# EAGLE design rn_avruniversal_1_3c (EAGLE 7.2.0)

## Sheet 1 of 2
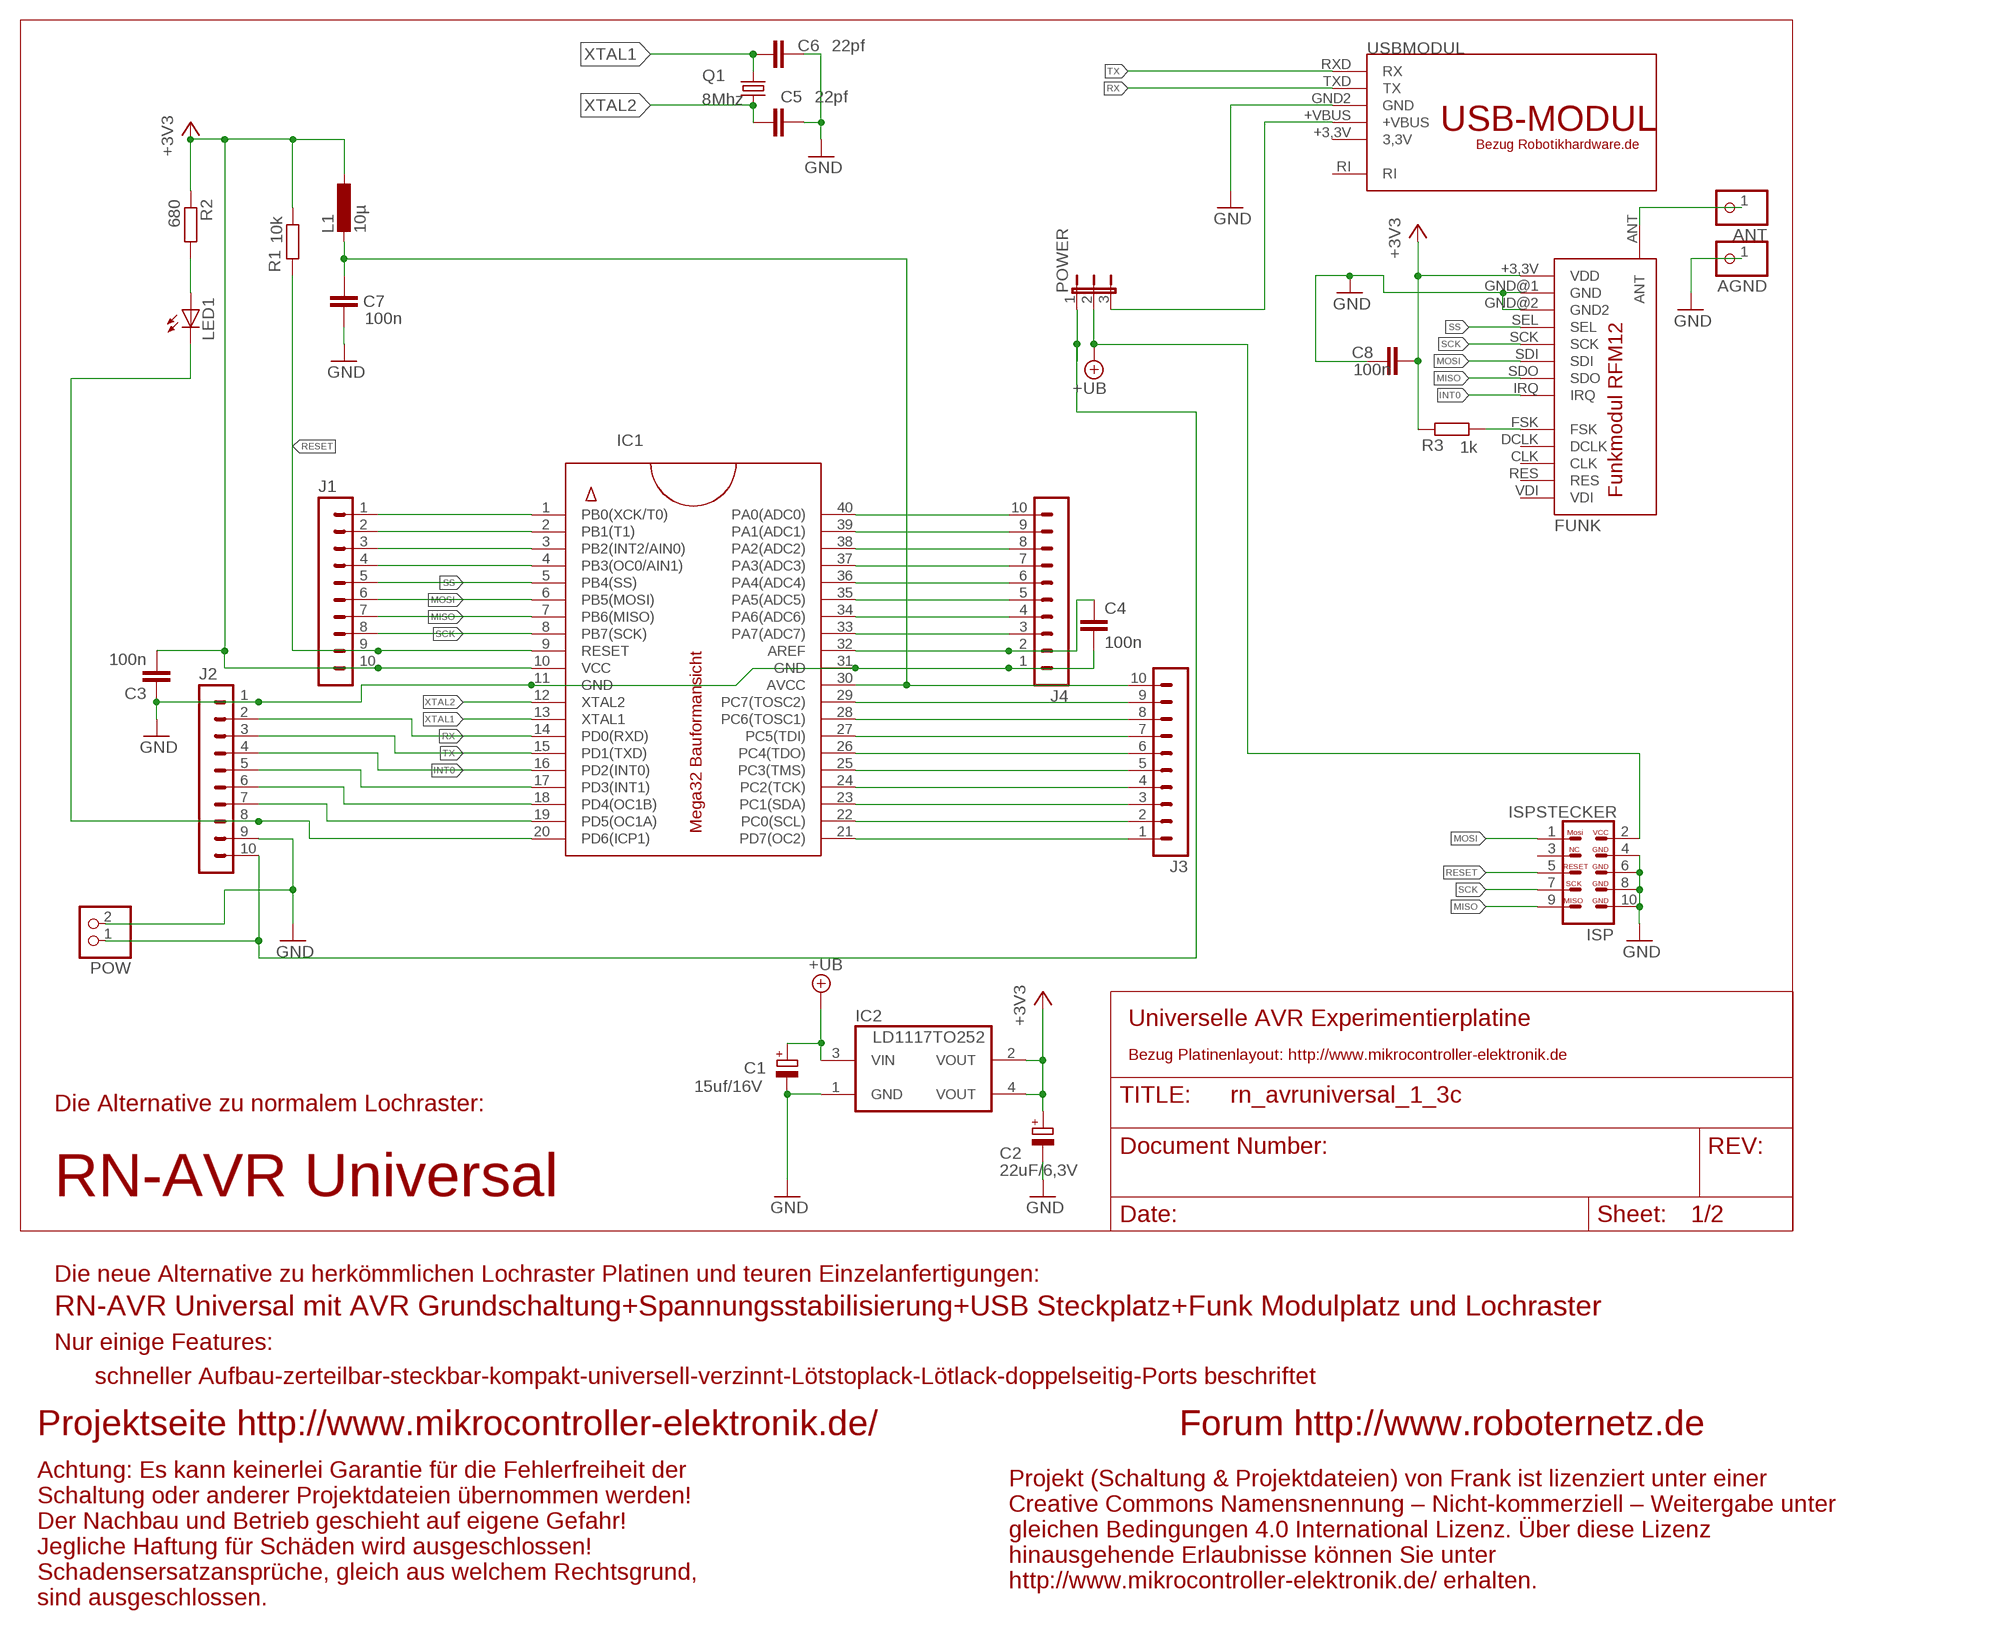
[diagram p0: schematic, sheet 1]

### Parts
AGND  PINHD-1X1  [1X01]
ANT  PINHD-1X1  [1X01]
C1  15uf/16V  CPOL-EUSMCC  [SMC_C]
C2  22uF/6,3V  CPOL-EUSMCC  [SMC_C]
C3  100n  C-EU050-024X044  [C050-024X044]
C4  100n  C-EU050-024X044  [C050-024X044]
C5  22pf  C-EU050-024X044  [C050-024X044]
C6  22pf  C-EU050-024X044  [C050-024X044]
C7  100n  C-EU050-024X044  [C050-024X044]
C8  100n  C-EU050-024X044  [C050-024X044]
FUNK  RFM12  [RFM12_SMD]
IC1  MEGA32BAUFORM  [DIL40]
IC2  LD1117TO252  [TO252]
ISP  ISPSTECKER  [ML10]
J1  AST021-10AST021-10PIN  [AST021-10PIN]
J2  AST021-10AST021-10PIN  [AST021-10PIN]
J3  AST021-10AST021-10PIN  [AST021-10PIN]
J4  AST021-10AST021-10PIN  [AST021-10PIN]
L1  10µ  L-EU0207/12  [0207/12]
LED1  LED3MM  [LED3MM]
POW  PINHD-1X2  [1X02]
POWER  JP2E  [JP2]
Q1  8Mhz  CRYTALHC49S  [HC49/S]
R1  10k  R-EU_0207/10  [0207/10]
R2  680  R-EU_0207/10  [0207/10]
R3  1k  R-EU_0207/10  [0207/10]
USBMODUL  USBMODUL_RN_BUCHSE  [USBMODUL_RN_STECKER]

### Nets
+3V3 [Power]: C2.+ C3.2 C8.2 FUNK.+3,3V(VDD) IC1.10(VCC) IC2.2(VOUT) IC2.4(VOUT) J1.10 L1.1 R1.1 R2.1 R3.2
+UB [Power]: C1.+ IC2.3(VIN) ISP.2 POWER.2
AREF: C4.1 IC1.32(AREF) J4.2
AVCC: C7.2 IC1.30(AVCC) J3.10 L1.2
GND [Power]: AGND.1 C1.- C2.- C3.1 C4.2 C5.1 C6.1 C7.1 C8.1 FUNK.GND@1(GND) FUNK.GND@2(GND2) IC1.11(GND) IC1.31(GND) IC2.1(GND) ISP.4 ISP.6 ISP.8 ISP.10 J2.1 J2.9 J4.1 POW.2 USBMODUL.GND2(GND)
INT0: FUNK.IRQ IC1.16(PD2(INT0)) J2.4
INT1: IC1.17(PD3(INT1)) J2.5
MISO: FUNK.SDO IC1.7(PB6(MISO)) ISP.9 J1.7
MOSI: FUNK.SDI IC1.6(PB5(MOSI)) ISP.1 J1.6
N$1: ANT.1 FUNK.ANT
N$2: FUNK.FSK R3.1
N$4 [Power]: POWER.3 USBMODUL.+VBUS
N$6: LED1.A R2.2
PA0: IC1.40(PA0(ADC0)) J4.10
PA1: IC1.39(PA1(ADC1)) J4.9
PA2: IC1.38(PA2(ADC2)) J4.8
PA3: IC1.37(PA3(ADC3)) J4.7
PA4: IC1.36(PA4(ADC4)) J4.6
PA5: IC1.35(PA5(ADC5)) J4.5
PA6: IC1.34(PA6(ADC6)) J4.4
PA7: IC1.33(PA7(ADC7)) J4.3
PB0: IC1.1(PB0(XCK/T0)) J1.1
PB1: IC1.2(PB1(T1)) J1.2
PB2: IC1.3(PB2(INT2/AIN0)) J1.3
PB3: IC1.4(PB3(OC0/AIN1)) J1.4
PC2: IC1.24(PC2(TCK)) J3.4
PC3: IC1.25(PC3(TMS)) J3.5
PC4: IC1.26(PC4(TDO)) J3.6
PC5: IC1.27(PC5(TDI)) J3.7
PC6: IC1.28(PC6(TOSC1)) J3.8
PC7: IC1.29(PC7(TOSC2)) J3.9
PD4: IC1.18(PD4(OC1B)) J2.6
PD5: IC1.19(PD5(OC1A)) J2.7
PD6: IC1.20(PD6(ICP1)) J2.8 LED1.K(C)
PD7: IC1.21(PD7(OC2)) J3.1
RESET: IC1.9(RESET) ISP.5 J1.9 R1.2
RX: IC1.14(PD0(RXD)) J2.2 USBMODUL.TXD(TX)
SCK: FUNK.SCK IC1.8(PB7(SCK)) ISP.7 J1.8
SCL: IC1.22(PC0(SCL)) J3.2
SDA: IC1.23(PC1(SDA)) J3.3
SS: FUNK.SEL IC1.5(PB4(SS)) J1.5
TX: IC1.15(PD1(TXD)) J2.3 USBMODUL.RXD(RX)
UEINGANG [Power]: J2.10 POW.1 POWER.1
XTAL1: C6.2 IC1.13(XTAL1) Q1.1
XTAL2: C5.2 IC1.12(XTAL2) Q1.2
Unconnected: FUNK.CLK FUNK.DCLK FUNK.RES FUNK.VDI ISP.3 USBMODUL.RI

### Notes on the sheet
- Universelle AVR Experimentierplatine
- Bezug Platinenlayout: http://www.mikrocontroller-elektronik.de
- Die Alternative zu normalem Lochraster:
- RN-AVR Universal
- Die neue Alternative zu herkömmlichen Lochraster Platinen und teuren Einzelanfertigungen:
- RN-AVR Universal mit AVR Grundschaltung+Spannungsstabilisierung+USB Steckplatz+Funk Modulplatz und Lochraster
- Nur einige Features:
- schneller Aufbau-zerteilbar-steckbar-kompakt-universell-verzinnt-Lötstoplack-Lötlack-doppelseitig-Ports beschriftet
- Projektseite http://www.mikrocontroller-elektronik.de/ | Forum http://www.roboternetz.de
- Projekt (Schaltung & Projektdateien) von Frank ist lizenziert unter einer
  Creative Commons Namensnennung – Nicht-kommerziell – Weitergabe unter
  gleichen Bedingungen 4.0 International Lizenz. Über diese Lizenz
  hinausgehende Erlaubnisse können Sie unter
  http://www.mikrocontroller-elektronik.de/ erhalten.
- Achtung: Es kann keinerlei Garantie für die Fehlerfreiheit der
  Schaltung oder anderer Projektdateien übernommen werden!
  Der Nachbau und Betrieb geschieht auf eigene Gefahr! 
  Jegliche Haftung für Schäden wird ausgeschlossen!
  Schadensersatzansprüche, gleich aus welchem Rechtsgrund,
  sind ausgeschlossen.

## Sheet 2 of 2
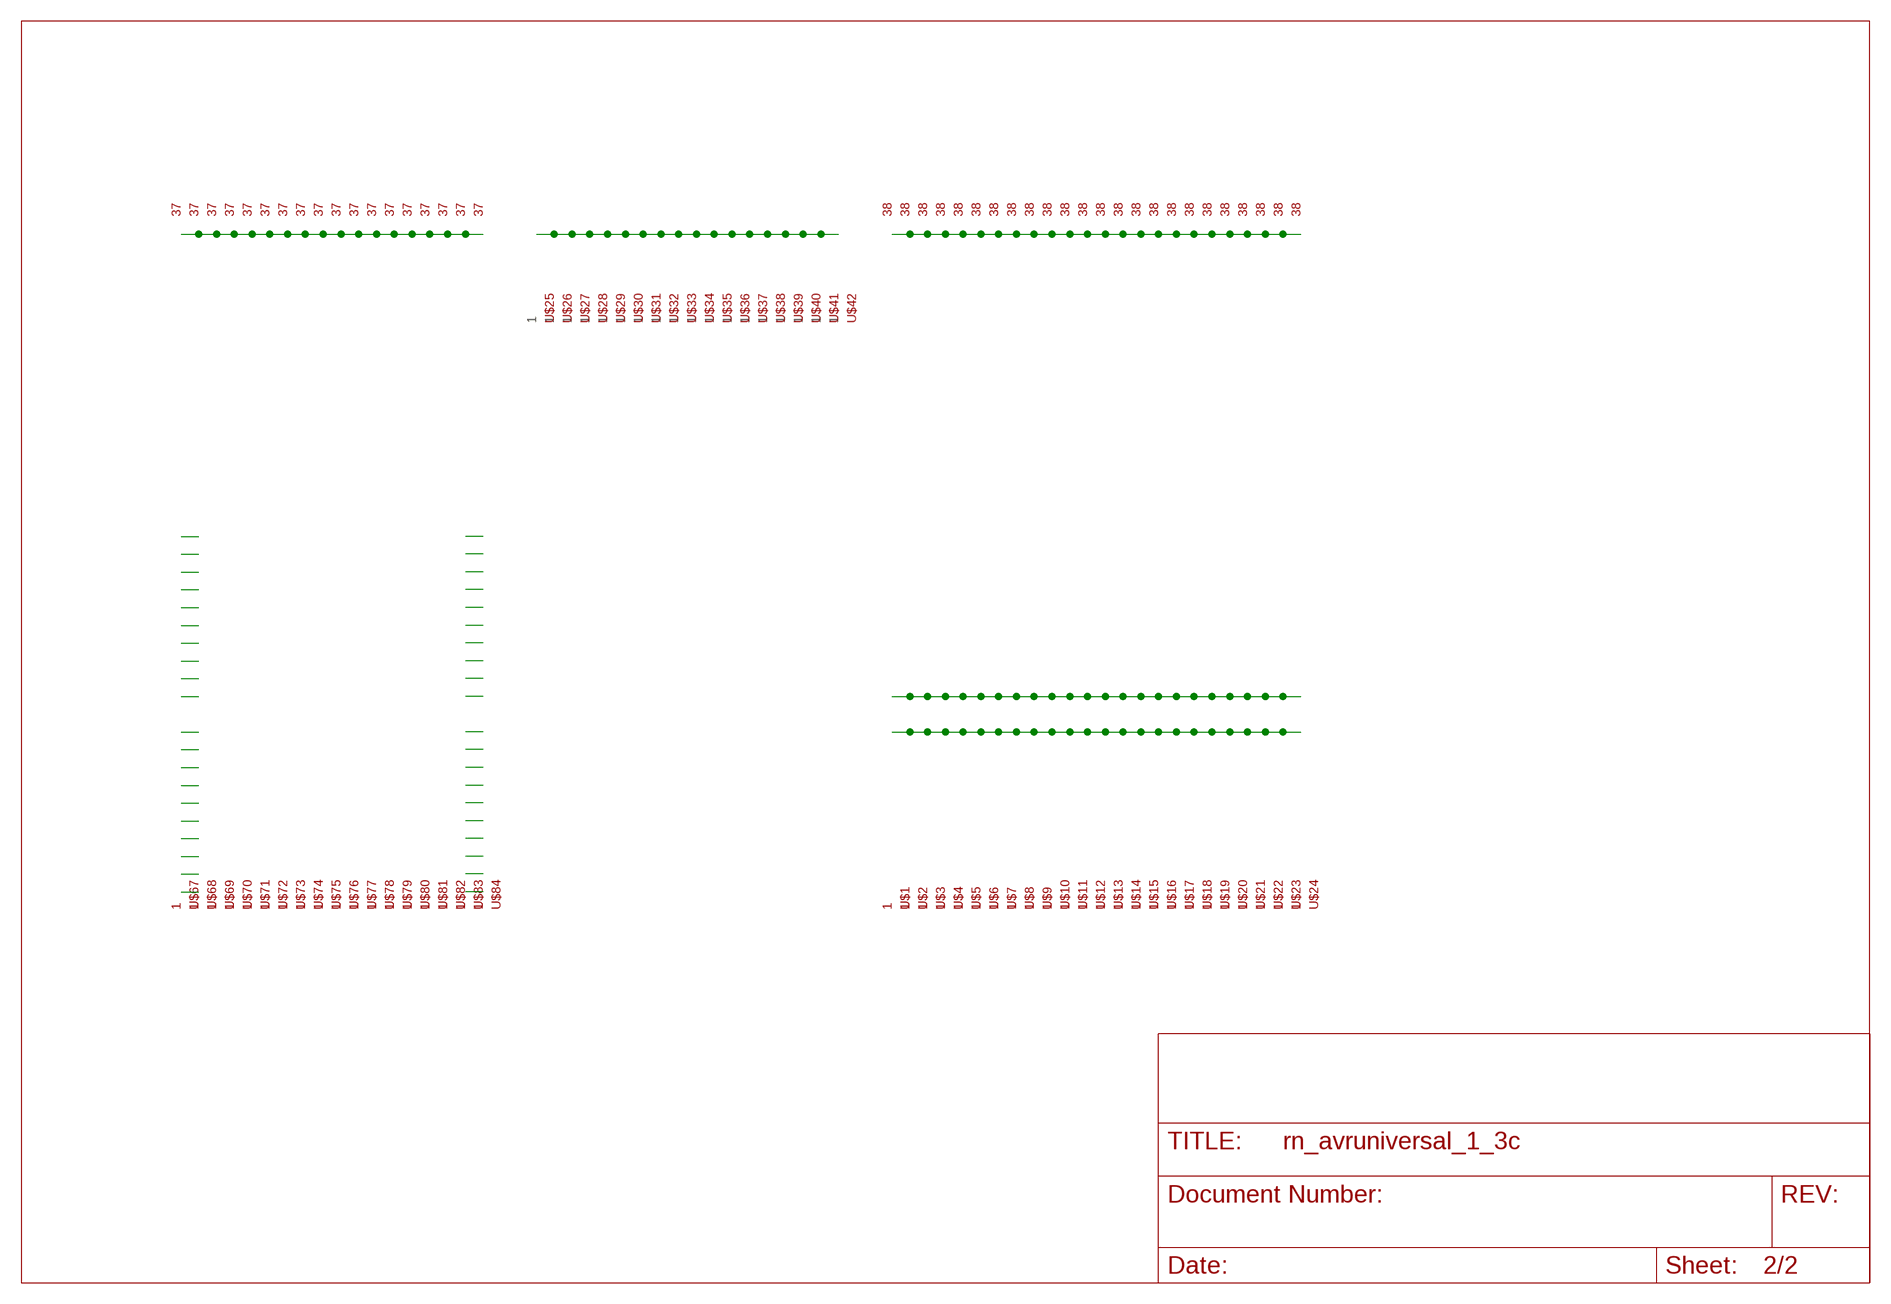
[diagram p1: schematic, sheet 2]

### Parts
U$1  LOCHRASTER38PIN  [LOCHRASTER38PIN]
U$2  LOCHRASTER38PIN  [LOCHRASTER38PIN]
U$3  LOCHRASTER38PIN  [LOCHRASTER38PIN]
U$4  LOCHRASTER38PIN  [LOCHRASTER38PIN]
U$5  LOCHRASTER38PIN  [LOCHRASTER38PIN]
U$6  LOCHRASTER38PIN  [LOCHRASTER38PIN]
U$7  LOCHRASTER38PIN  [LOCHRASTER38PIN]
U$8  LOCHRASTER38PIN  [LOCHRASTER38PIN]
U$9  LOCHRASTER38PIN  [LOCHRASTER38PIN]
U$10  LOCHRASTER38PIN  [LOCHRASTER38PIN]
U$11  LOCHRASTER38PIN  [LOCHRASTER38PIN]
U$12  LOCHRASTER38PIN  [LOCHRASTER38PIN]
U$13  LOCHRASTER38PIN  [LOCHRASTER38PIN]
U$14  LOCHRASTER38PIN  [LOCHRASTER38PIN]
U$15  LOCHRASTER38PIN  [LOCHRASTER38PIN]
U$16  LOCHRASTER38PIN  [LOCHRASTER38PIN]
U$17  LOCHRASTER38PIN  [LOCHRASTER38PIN]
U$18  LOCHRASTER38PIN  [LOCHRASTER38PIN]
U$19  LOCHRASTER38PIN  [LOCHRASTER38PIN]
U$20  LOCHRASTER38PIN  [LOCHRASTER38PIN]
U$21  LOCHRASTER38PIN  [LOCHRASTER38PIN]
U$22  LOCHRASTER38PIN  [LOCHRASTER38PIN]
U$23  LOCHRASTER38PIN  [LOCHRASTER38PIN]
U$24  LOCHRASTER38PIN  [LOCHRASTER38PIN]
U$25  LOCHRASTER5PIN  [LOACHRASTER5PIN]
U$26  LOCHRASTER5PIN  [LOACHRASTER5PIN]
U$27  LOCHRASTER5PIN  [LOACHRASTER5PIN]
U$28  LOCHRASTER5PIN  [LOACHRASTER5PIN]
U$29  LOCHRASTER5PIN  [LOACHRASTER5PIN]
U$30  LOCHRASTER5PIN  [LOACHRASTER5PIN]
U$31  LOCHRASTER5PIN  [LOACHRASTER5PIN]
U$32  LOCHRASTER5PIN  [LOACHRASTER5PIN]
U$33  LOCHRASTER5PIN  [LOACHRASTER5PIN]
U$34  LOCHRASTER5PIN  [LOACHRASTER5PIN]
U$35  LOCHRASTER5PIN  [LOACHRASTER5PIN]
U$36  LOCHRASTER5PIN  [LOACHRASTER5PIN]
U$37  LOCHRASTER5PIN  [LOACHRASTER5PIN]
U$38  LOCHRASTER5PIN  [LOACHRASTER5PIN]
U$39  LOCHRASTER5PIN  [LOACHRASTER5PIN]
U$40  LOCHRASTER5PIN  [LOACHRASTER5PIN]
U$41  LOCHRASTER5PIN  [LOACHRASTER5PIN]
U$42  LOCHRASTER5PIN  [LOACHRASTER5PIN]
U$67  LOCHRASTER37PIN  [LOCHRASTER37PIN]
U$68  LOCHRASTER37PIN  [LOCHRASTER37PIN]
U$69  LOCHRASTER37PIN  [LOCHRASTER37PIN]
U$70  LOCHRASTER37PIN  [LOCHRASTER37PIN]
U$71  LOCHRASTER37PIN  [LOCHRASTER37PIN]
U$72  LOCHRASTER37PIN  [LOCHRASTER37PIN]
U$73  LOCHRASTER37PIN  [LOCHRASTER37PIN]
U$74  LOCHRASTER37PIN  [LOCHRASTER37PIN]
U$75  LOCHRASTER37PIN  [LOCHRASTER37PIN]
U$76  LOCHRASTER37PIN  [LOCHRASTER37PIN]
U$77  LOCHRASTER37PIN  [LOCHRASTER37PIN]
U$78  LOCHRASTER37PIN  [LOCHRASTER37PIN]
U$79  LOCHRASTER37PIN  [LOCHRASTER37PIN]
U$80  LOCHRASTER37PIN  [LOCHRASTER37PIN]
U$81  LOCHRASTER37PIN  [LOCHRASTER37PIN]
U$82  LOCHRASTER37PIN  [LOCHRASTER37PIN]
U$83  LOCHRASTER37PIN  [LOCHRASTER37PIN]
U$84  LOCHRASTER37PIN  [LOCHRASTER37PIN]

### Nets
N$3 [SuperPower]: U$1.P$10 U$2.P$10 U$3.P$10 U$4.P$10 U$5.P$10 U$6.P$10 U$7.P$10 U$8.P$10 U$9.P$10 U$10.P$10 U$11.P$10 U$12.P$10 U$13.P$10 U$14.P$10 U$15.P$10 U$16.P$10 U$17.P$10 U$18.P$10 U$19.P$10 U$20.P$10 U$21.P$10 U$22.P$10 U$23.P$10 U$24.P$10
N$7 [Dick]: U$83.P$1 U$84.P$1
N$8 [Dick]: U$83.P$2 U$84.P$2
N$9 [SuperPower]: U$1.P$12 U$2.P$12 U$3.P$12 U$4.P$12 U$5.P$12 U$6.P$12 U$7.P$12 U$8.P$12 U$9.P$12 U$10.P$12 U$11.P$12 U$12.P$12 U$13.P$12 U$14.P$12 U$15.P$12 U$16.P$12 U$17.P$12 U$18.P$12 U$19.P$12 U$20.P$12 U$21.P$12 U$22.P$12 U$23.P$12 U$24.P$12
N$10 [Dick]: U$83.P$3 U$84.P$3
N$11 [Dick]: U$83.P$4 U$84.P$4
N$12 [Dick]: U$83.P$5 U$84.P$5
N$13 [Dick]: U$83.P$6 U$84.P$6
N$14 [Dick]: U$83.P$7 U$84.P$7
N$15 [Dick]: U$83.P$8 U$84.P$8
N$16 [Dick]: U$83.P$9 U$84.P$9
N$17 [Dick]: U$83.P$10 U$84.P$10
N$18 [Dick]: U$83.P$12 U$84.P$12
N$19 [Dick]: U$83.P$13 U$84.P$13
N$20 [Dick]: U$83.P$14 U$84.P$14
N$21 [SuperPower]: U$67.37 U$68.37 U$69.37 U$70.37 U$71.37 U$72.37 U$73.37 U$74.37 U$75.37 U$76.37 U$77.37 U$78.37 U$79.37 U$80.37 U$81.37 U$82.37 U$83.37 U$84.37
N$22 [Dick]: U$83.P$15 U$84.P$15
N$23 [Dick]: U$83.P$16 U$84.P$16
N$24 [Dick]: U$83.P$17 U$84.P$17
N$25: U$25.5 U$26.5 U$27.5 U$28.5 U$29.5 U$30.5 U$31.5 U$32.5 U$33.5 U$34.5 U$35.5 U$36.5 U$37.5 U$38.5 U$39.5 U$40.5 U$41.5 U$42.5
N$26 [Dick]: U$83.P$18 U$84.P$18
N$27: U$83.P$19 U$84.P$19
N$28 [SuperPower]: U$1.P$38 U$2.P$38 U$3.P$38 U$4.P$38 U$5.P$38 U$6.P$38 U$7.P$38 U$8.P$38 U$9.P$38 U$10.P$38 U$11.P$38 U$12.P$38 U$13.P$38 U$14.P$38 U$15.P$38 U$16.P$38 U$17.P$38 U$18.P$38 U$19.P$38 U$20.P$38 U$21.P$38 U$22.P$38 U$23.P$38 U$24.P$38
N$29: U$83.P$20 U$84.P$20
N$30: U$83.P$21 U$84.P$21
N$31 [Dick]: U$67.P$1 U$68.P$1
N$32 [Dick]: U$67.P$2 U$68.P$2
N$33 [Dick]: U$67.P$3 U$68.P$3
N$34 [Dick]: U$67.P$4 U$68.P$4
N$35 [Dick]: U$67.P$5 U$68.P$5
N$36 [Dick]: U$67.P$6 U$68.P$6
N$37 [Dick]: U$67.P$7 U$68.P$7
N$38 [Dick]: U$67.P$8 U$68.P$8
N$39 [Dick]: U$67.P$9 U$68.P$9
N$40 [Dick]: U$67.P$10 U$68.P$10
N$41 [Dick]: U$67.P$12 U$68.P$12
N$42 [Dick]: U$67.P$13 U$68.P$13
N$43 [Dick]: U$67.P$14 U$68.P$14
N$44 [Dick]: U$67.P$15 U$68.P$15
N$45 [Dick]: U$67.P$16 U$68.P$16
N$46 [Dick]: U$67.P$17 U$68.P$17
N$47 [Dick]: U$67.P$18 U$68.P$18
N$48 [Dick]: U$67.P$19 U$68.P$19
N$49 [Dick]: U$67.P$20 U$68.P$20
N$50 [Dick]: U$67.P$21 U$68.P$21
Unconnected: U$1.P$1 U$1.P$2 U$1.P$3 U$1.P$4 U$1.P$5 U$1.P$6 U$1.P$7 U$1.P$8 U$1.P$9 U$1.P$11 U$1.P$13 U$1.P$14 U$1.P$15 U$1.P$16 U$1.P$17 U$1.P$18 U$1.P$19 U$1.P$20 U$1.P$21 U$1.P$22 U$1.P$23 U$1.P$24 U$1.P$25 U$1.P$26 U$1.P$27 U$1.P$28 U$1.P$29 U$1.P$30 U$1.P$31 U$1.P$32 U$1.P$33 U$1.P$34 U$1.P$35 U$1.P$36 U$1.P$37 U$2.P$1 U$2.P$2 U$2.P$3 U$2.P$4 U$2.P$5 U$2.P$6 U$2.P$7 U$2.P$8 U$2.P$9 U$2.P$11 U$2.P$13 U$2.P$14 U$2.P$15 U$2.P$16 U$2.P$17 U$2.P$18 U$2.P$19 U$2.P$20 U$2.P$21 U$2.P$22 U$2.P$23 U$2.P$24 U$2.P$25 U$2.P$26 U$2.P$27 U$2.P$28 U$2.P$29 U$2.P$30 U$2.P$31 U$2.P$32 U$2.P$33 U$2.P$34 U$2.P$35 U$2.P$36 U$2.P$37 U$3.P$1 U$3.P$2 U$3.P$3 U$3.P$4 U$3.P$5 U$3.P$6 U$3.P$7 U$3.P$8 U$3.P$9 U$3.P$11 U$3.P$13 U$3.P$14 U$3.P$15 U$3.P$16 U$3.P$17 U$3.P$18 U$3.P$19 U$3.P$20 U$3.P$21 U$3.P$22 U$3.P$23 U$3.P$24 U$3.P$25 U$3.P$26 U$3.P$27 U$3.P$28 U$3.P$29 U$3.P$30 U$3.P$31 U$3.P$32 U$3.P$33 U$3.P$34 U$3.P$35 U$3.P$36 U$3.P$37 U$4.P$1 U$4.P$2 U$4.P$3 U$4.P$4 U$4.P$5 U$4.P$6 U$4.P$7 U$4.P$8 U$4.P$9 U$4.P$11 U$4.P$13 U$4.P$14 U$4.P$15 U$4.P$16 U$4.P$17 U$4.P$18 U$4.P$19 U$4.P$20 U$4.P$21 U$4.P$22 U$4.P$23 U$4.P$24 U$4.P$25 U$4.P$26 U$4.P$27 U$4.P$28 U$4.P$29 U$4.P$30 U$4.P$31 U$4.P$32 U$4.P$33 U$4.P$34 U$4.P$35 U$4.P$36 U$4.P$37 U$5.P$1 U$5.P$2 U$5.P$3 U$5.P$4 U$5.P$5 U$5.P$6 U$5.P$7 U$5.P$8 U$5.P$9 U$5.P$11 U$5.P$13 U$5.P$14 U$5.P$15 U$5.P$16 U$5.P$17 U$5.P$18 U$5.P$19 U$5.P$20 U$5.P$21 U$5.P$22 U$5.P$23 U$5.P$24 U$5.P$25 U$5.P$26 U$5.P$27 U$5.P$28 U$5.P$29 U$5.P$30 U$5.P$31 U$5.P$32 U$5.P$33 U$5.P$34 U$5.P$35 U$5.P$36 U$5.P$37 U$6.P$1 U$6.P$2 U$6.P$3 U$6.P$4 U$6.P$5 U$6.P$6 U$6.P$7 U$6.P$8 U$6.P$9 U$6.P$11 U$6.P$13 U$6.P$14 U$6.P$15 U$6.P$16 U$6.P$17 U$6.P$18 U$6.P$19 U$6.P$20 U$6.P$21 U$6.P$22 U$6.P$23 U$6.P$24 U$6.P$25 U$6.P$26 U$6.P$27 U$6.P$28 U$6.P$29 U$6.P$30 U$6.P$31 U$6.P$32 U$6.P$33 U$6.P$34 U$6.P$35 U$6.P$36 U$6.P$37 U$7.P$1 U$7.P$2 U$7.P$3 U$7.P$4 U$7.P$5 U$7.P$6 U$7.P$7 U$7.P$8 U$7.P$9 U$7.P$11 U$7.P$13 U$7.P$14 U$7.P$15 U$7.P$16 U$7.P$17 U$7.P$18 U$7.P$19 U$7.P$20 U$7.P$21 U$7.P$22 U$7.P$23 U$7.P$24 U$7.P$25 U$7.P$26 U$7.P$27 U$7.P$28 U$7.P$29 U$7.P$30 U$7.P$31 U$7.P$32 U$7.P$33 U$7.P$34 U$7.P$35 U$7.P$36 U$7.P$37 U$8.P$1 U$8.P$2 U$8.P$3 U$8.P$4 U$8.P$5 U$8.P$6 U$8.P$7 U$8.P$8 U$8.P$9 U$8.P$11 U$8.P$13 U$8.P$14 U$8.P$15 U$8.P$16 U$8.P$17 U$8.P$18 U$8.P$19 U$8.P$20 U$8.P$21 U$8.P$22 U$8.P$23 U$8.P$24 U$8.P$25 U$8.P$26 U$8.P$27 U$8.P$28 U$8.P$29 U$8.P$30 U$8.P$31 U$8.P$32 U$8.P$33 U$8.P$34 U$8.P$35 U$8.P$36 U$8.P$37 U$9.P$1 U$9.P$2 U$9.P$3 U$9.P$4 U$9.P$5 U$9.P$6 U$9.P$7 U$9.P$8 U$9.P$9 U$9.P$11 U$9.P$13 U$9.P$14 U$9.P$15 U$9.P$16 U$9.P$17 U$9.P$18 U$9.P$19 U$9.P$20 U$9.P$21 U$9.P$22 U$9.P$23 U$9.P$24 U$9.P$25 U$9.P$26 U$9.P$27 U$9.P$28 U$9.P$29 U$9.P$30 U$9.P$31 U$9.P$32 U$9.P$33 U$9.P$34 U$9.P$35 U$9.P$36 U$9.P$37 U$10.P$1 U$10.P$2 U$10.P$3 U$10.P$4 U$10.P$5 U$10.P$6 U$10.P$7 U$10.P$8 U$10.P$9 U$10.P$11 U$10.P$13 U$10.P$14 U$10.P$15 U$10.P$16 U$10.P$17 U$10.P$18 U$10.P$19 U$10.P$20 U$10.P$21 U$10.P$22 U$10.P$23 U$10.P$24 U$10.P$25 U$10.P$26 U$10.P$27 U$10.P$28 U$10.P$29 U$10.P$30 U$10.P$31 U$10.P$32 U$10.P$33 U$10.P$34 U$10.P$35 U$10.P$36 U$10.P$37 U$11.P$1 U$11.P$2 U$11.P$3 U$11.P$4 U$11.P$5 U$11.P$6 U$11.P$7 U$11.P$8 U$11.P$9 U$11.P$11 U$11.P$13 U$11.P$14 U$11.P$15 U$11.P$16 U$11.P$17 U$11.P$18 U$11.P$19 U$11.P$20 U$11.P$21 U$11.P$22 U$11.P$23 U$11.P$24 U$11.P$25 U$11.P$26 U$11.P$27 U$11.P$28 U$11.P$29 U$11.P$30 U$11.P$31 U$11.P$32 U$11.P$33 U$11.P$34 U$11.P$35 U$11.P$36 U$11.P$37 U$12.P$1 U$12.P$2 U$12.P$3 U$12.P$4 U$12.P$5 U$12.P$6 U$12.P$7 U$12.P$8 U$12.P$9 U$12.P$11 U$12.P$13 U$12.P$14 U$12.P$15 U$12.P$16 U$12.P$17 U$12.P$18 U$12.P$19 U$12.P$20 U$12.P$21 U$12.P$22 U$12.P$23 U$12.P$24 U$12.P$25 U$12.P$26 U$12.P$27 U$12.P$28 U$12.P$29 U$12.P$30 U$12.P$31 U$12.P$32 U$12.P$33 U$12.P$34 U$12.P$35 U$12.P$36 U$12.P$37 U$13.P$1 U$13.P$2 U$13.P$3 U$13.P$4 U$13.P$5 U$13.P$6 U$13.P$7 U$13.P$8 U$13.P$9 U$13.P$11 U$13.P$13 U$13.P$14 U$13.P$15 U$13.P$16 U$13.P$17 U$13.P$18 U$13.P$19 U$13.P$20 U$13.P$21 U$13.P$22 U$13.P$23 U$13.P$24 U$13.P$25 U$13.P$26 U$13.P$27 U$13.P$28 U$13.P$29 U$13.P$30 U$13.P$31 U$13.P$32 U$13.P$33 U$13.P$34 U$13.P$35 U$13.P$36 U$13.P$37 U$14.P$1 U$14.P$2 U$14.P$3 U$14.P$4 U$14.P$5 U$14.P$6 U$14.P$7 U$14.P$8 U$14.P$9 U$14.P$11 U$14.P$13 U$14.P$14 U$14.P$15 U$14.P$16 U$14.P$17 U$14.P$18 U$14.P$19 U$14.P$20 U$14.P$21 U$14.P$22 U$14.P$23 U$14.P$24 U$14.P$25 U$14.P$26 U$14.P$27 U$14.P$28 U$14.P$29 U$14.P$30 U$14.P$31 U$14.P$32 U$14.P$33 U$14.P$34 U$14.P$35 U$14.P$36 U$14.P$37 U$15.P$1 U$15.P$2 U$15.P$3 U$15.P$4 U$15.P$5 U$15.P$6 U$15.P$7 U$15.P$8 U$15.P$9 U$15.P$11 U$15.P$13 U$15.P$14 U$15.P$15 U$15.P$16 U$15.P$17 U$15.P$18 U$15.P$19 U$15.P$20 U$15.P$21 U$15.P$22 U$15.P$23 U$15.P$24 U$15.P$25 U$15.P$26 U$15.P$27 U$15.P$28 U$15.P$29 U$15.P$30 U$15.P$31 U$15.P$32 U$15.P$33 U$15.P$34 U$15.P$35 U$15.P$36 U$15.P$37 U$16.P$1 U$16.P$2 U$16.P$3 U$16.P$4 U$16.P$5 U$16.P$6 U$16.P$7 U$16.P$8 U$16.P$9 U$16.P$11 U$16.P$13 U$16.P$14 U$16.P$15 U$16.P$16 U$16.P$17 U$16.P$18 U$16.P$19 U$16.P$20 U$16.P$21 U$16.P$22 U$16.P$23 U$16.P$24 U$16.P$25 U$16.P$26 U$16.P$27 U$16.P$28 U$16.P$29 U$16.P$30 U$16.P$31 U$16.P$32 U$16.P$33 U$16.P$34 U$16.P$35 U$16.P$36 U$16.P$37 U$17.P$1 U$17.P$2 U$17.P$3 U$17.P$4 U$17.P$5 U$17.P$6 U$17.P$7 U$17.P$8 U$17.P$9 U$17.P$11 U$17.P$13 U$17.P$14 U$17.P$15 U$17.P$16 U$17.P$17 U$17.P$18 U$17.P$19 U$17.P$20 U$17.P$21 U$17.P$22 U$17.P$23 U$17.P$24 U$17.P$25 U$17.P$26 U$17.P$27 U$17.P$28 U$17.P$29 U$17.P$30 U$17.P$31 U$17.P$32 U$17.P$33 U$17.P$34 U$17.P$35 U$17.P$36 U$17.P$37 U$18.P$1 U$18.P$2 U$18.P$3 U$18.P$4 U$18.P$5 U$18.P$6 U$18.P$7 U$18.P$8 U$18.P$9 U$18.P$11 U$18.P$13 U$18.P$14 U$18.P$15 U$18.P$16 U$18.P$17 U$18.P$18 U$18.P$19 U$18.P$20 U$18.P$21 U$18.P$22 U$18.P$23 U$18.P$24 U$18.P$25 U$18.P$26 U$18.P$27 U$18.P$28 U$18.P$29 U$18.P$30 U$18.P$31 U$18.P$32 U$18.P$33 U$18.P$34 U$18.P$35 U$18.P$36 U$18.P$37 U$19.P$1 U$19.P$2 U$19.P$3 U$19.P$4 U$19.P$5 U$19.P$6 U$19.P$7 U$19.P$8 U$19.P$9 U$19.P$11 U$19.P$13 U$19.P$14 U$19.P$15 U$19.P$16 U$19.P$17 U$19.P$18 U$19.P$19 U$19.P$20 U$19.P$21 U$19.P$22 U$19.P$23 U$19.P$24 U$19.P$25 U$19.P$26 U$19.P$27 U$19.P$28 U$19.P$29 U$19.P$30 U$19.P$31 U$19.P$32 U$19.P$33 U$19.P$34 U$19.P$35 U$19.P$36 U$19.P$37 U$20.P$1 U$20.P$2 U$20.P$3 U$20.P$4 U$20.P$5 U$20.P$6 U$20.P$7 U$20.P$8 U$20.P$9 U$20.P$11 U$20.P$13 U$20.P$14 U$20.P$15 U$20.P$16 U$20.P$17 U$20.P$18 U$20.P$19 U$20.P$20 U$20.P$21 U$20.P$22 U$20.P$23 U$20.P$24 U$20.P$25 U$20.P$26 U$20.P$27 U$20.P$28 U$20.P$29 U$20.P$30 U$20.P$31 U$20.P$32 U$20.P$33 U$20.P$34 U$20.P$35 U$20.P$36 U$20.P$37 U$21.P$1 U$21.P$2 U$21.P$3 U$21.P$4 U$21.P$5 U$21.P$6 U$21.P$7 U$21.P$8 U$21.P$9 U$21.P$11 U$21.P$13 U$21.P$14 U$21.P$15 U$21.P$16 U$21.P$17 U$21.P$18 U$21.P$19 U$21.P$20 U$21.P$21 U$21.P$22 U$21.P$23 U$21.P$24 U$21.P$25 U$21.P$26 U$21.P$27 U$21.P$28 U$21.P$29 U$21.P$30 U$21.P$31 U$21.P$32 U$21.P$33 U$21.P$34 U$21.P$35 U$21.P$36 U$21.P$37 U$22.P$1 U$22.P$2 U$22.P$3 U$22.P$4 U$22.P$5 U$22.P$6 U$22.P$7 U$22.P$8 U$22.P$9 U$22.P$11 U$22.P$13 U$22.P$14 U$22.P$15 U$22.P$16 U$22.P$17 U$22.P$18 U$22.P$19 U$22.P$20 U$22.P$21 U$22.P$22 U$22.P$23 U$22.P$24 U$22.P$25 U$22.P$26 U$22.P$27 U$22.P$28 U$22.P$29 U$22.P$30 U$22.P$31 U$22.P$32 U$22.P$33 U$22.P$34 U$22.P$35 U$22.P$36 U$22.P$37 U$23.P$1 U$23.P$2 U$23.P$3 U$23.P$4 U$23.P$5 U$23.P$6 U$23.P$7 U$23.P$8 U$23.P$9 U$23.P$11 U$23.P$13 U$23.P$14 U$23.P$15 U$23.P$16 U$23.P$17 U$23.P$18 U$23.P$19 U$23.P$20 U$23.P$21 U$23.P$22 U$23.P$23 U$23.P$24 U$23.P$25 U$23.P$26 U$23.P$27 U$23.P$28 U$23.P$29 U$23.P$30 U$23.P$31 U$23.P$32 U$23.P$33 U$23.P$34 U$23.P$35 U$23.P$36 U$23.P$37 U$24.P$1 U$24.P$2 U$24.P$3 U$24.P$4 U$24.P$5 U$24.P$6 U$24.P$7 U$24.P$8 U$24.P$9 U$24.P$11 U$24.P$13 U$24.P$14 U$24.P$15 U$24.P$16 U$24.P$17 U$24.P$18 U$24.P$19 U$24.P$20 U$24.P$21 U$24.P$22 U$24.P$23 U$24.P$24 U$24.P$25 U$24.P$26 U$24.P$27 U$24.P$28 U$24.P$29 U$24.P$30 U$24.P$31 U$24.P$32 U$24.P$33 U$24.P$34 U$24.P$35 U$24.P$36 U$24.P$37 U$25.1 U$25.2 U$25.3 U$25.4 U$26.1 U$26.2 U$26.3 U$26.4 U$27.1 U$27.2 U$27.3 U$27.4 U$28.1 U$28.2 U$28.3 U$28.4 U$29.1 U$29.2 U$29.3 U$29.4 U$30.1 U$30.2 U$30.3 U$30.4 U$31.1 U$31.2 U$31.3 U$31.4 U$32.1 U$32.2 U$32.3 U$32.4 U$33.1 U$33.2 U$33.3 U$33.4 U$34.1 U$34.2 U$34.3 U$34.4 U$35.1 U$35.2 U$35.3 U$35.4 U$36.1 U$36.2 U$36.3 U$36.4 U$37.1 U$37.2 U$37.3 U$37.4 U$38.1 U$38.2 U$38.3 U$38.4 U$39.1 U$39.2 U$39.3 U$39.4 U$40.1 U$40.2 U$40.3 U$40.4 U$41.1 U$41.2 U$41.3 U$41.4 U$42.1 U$42.2 U$42.3 U$42.4 U$67.33 U$67.34 U$67.35 U$67.36 U$67.P$11 U$67.P$22 U$67.P$23 U$67.P$24 U$67.P$25 U$67.P$26 U$67.P$27 U$67.P$28 U$67.P$29 U$67.P$30 U$67.P$31 U$67.P$32 U$68.33 U$68.34 U$68.35 U$68.36 U$68.P$11 U$68.P$22 U$68.P$23 U$68.P$24 U$68.P$25 U$68.P$26 U$68.P$27 U$68.P$28 U$68.P$29 U$68.P$30 U$68.P$31 U$68.P$32 U$69.33 U$69.34 U$69.35 U$69.36 U$69.P$1 U$69.P$2 U$69.P$3 U$69.P$4 U$69.P$5 U$69.P$6 U$69.P$7 U$69.P$8 U$69.P$9 U$69.P$10 U$69.P$11 U$69.P$12 U$69.P$13 U$69.P$14 U$69.P$15 U$69.P$16 U$69.P$17 U$69.P$18 U$69.P$19 U$69.P$20 U$69.P$21 U$69.P$22 U$69.P$23 U$69.P$24 U$69.P$25 U$69.P$26 U$69.P$27 U$69.P$28 U$69.P$29 U$69.P$30 U$69.P$31 U$69.P$32 U$70.33 U$70.34 U$70.35 U$70.36 U$70.P$1 U$70.P$2 U$70.P$3 U$70.P$4 U$70.P$5 U$70.P$6 U$70.P$7 U$70.P$8 U$70.P$9 U$70.P$10 U$70.P$11 U$70.P$12 U$70.P$13 U$70.P$14 U$70.P$15 U$70.P$16 U$70.P$17 U$70.P$18 U$70.P$19 U$70.P$20 U$70.P$21 U$70.P$22 U$70.P$23 U$70.P$24 U$70.P$25 U$70.P$26 U$70.P$27 U$70.P$28 U$70.P$29 U$70.P$30 U$70.P$31 U$70.P$32 U$71.33 U$71.34 U$71.35 U$71.36 U$71.P$1 U$71.P$2 U$71.P$3 U$71.P$4 U$71.P$5 U$71.P$6 U$71.P$7 U$71.P$8 U$71.P$9 U$71.P$10 U$71.P$11 U$71.P$12 U$71.P$13 U$71.P$14 U$71.P$15 U$71.P$16 U$71.P$17 U$71.P$18 U$71.P$19 U$71.P$20 U$71.P$21 U$71.P$22 U$71.P$23 U$71.P$24 U$71.P$25 U$71.P$26 U$71.P$27 U$71.P$28 U$71.P$29 U$71.P$30 U$71.P$31 U$71.P$32 U$72.33 U$72.34 U$72.35 U$72.36 U$72.P$1 U$72.P$2 U$72.P$3 U$72.P$4 U$72.P$5 U$72.P$6 U$72.P$7 U$72.P$8 U$72.P$9 U$72.P$10 U$72.P$11 U$72.P$12 U$72.P$13 U$72.P$14 U$72.P$15 U$72.P$16 U$72.P$17 U$72.P$18 U$72.P$19 U$72.P$20 U$72.P$21 U$72.P$22 U$72.P$23 U$72.P$24 U$72.P$25 U$72.P$26 U$72.P$27 U$72.P$28 U$72.P$29 U$72.P$30 U$72.P$31 U$72.P$32 U$73.33 U$73.34 U$73.35 U$73.36 U$73.P$1 U$73.P$2 U$73.P$3 U$73.P$4 U$73.P$5 U$73.P$6 U$73.P$7 U$73.P$8 U$73.P$9 U$73.P$10 U$73.P$11 U$73.P$12 U$73.P$13 U$73.P$14 U$73.P$15 U$73.P$16 U$73.P$17 U$73.P$18 U$73.P$19 U$73.P$20 U$73.P$21 U$73.P$22 U$73.P$23 U$73.P$24 U$73.P$25 U$73.P$26 U$73.P$27 U$73.P$28 U$73.P$29 U$73.P$30 U$73.P$31 U$73.P$32 U$74.33 U$74.34 U$74.35 U$74.36 U$74.P$1 U$74.P$2 U$74.P$3 U$74.P$4 U$74.P$5 U$74.P$6 U$74.P$7 U$74.P$8 U$74.P$9 U$74.P$10 U$74.P$11 U$74.P$12 U$74.P$13 U$74.P$14 U$74.P$15 U$74.P$16 U$74.P$17 U$74.P$18 U$74.P$19 U$74.P$20 U$74.P$21 U$74.P$22 U$74.P$23 U$74.P$24 U$74.P$25 U$74.P$26 U$74.P$27 U$74.P$28 U$74.P$29 U$74.P$30 U$74.P$31 U$74.P$32 U$75.33 U$75.34 U$75.35 U$75.36 U$75.P$1 U$75.P$2 U$75.P$3 U$75.P$4 U$75.P$5 U$75.P$6 U$75.P$7 U$75.P$8 U$75.P$9 U$75.P$10 U$75.P$11 U$75.P$12 U$75.P$13 U$75.P$14 U$75.P$15 U$75.P$16 U$75.P$17 U$75.P$18 U$75.P$19 U$75.P$20 U$75.P$21 U$75.P$22 U$75.P$23 U$75.P$24 U$75.P$25 U$75.P$26 U$75.P$27 U$75.P$28 U$75.P$29 U$75.P$30 U$75.P$31 U$75.P$32 U$76.33 U$76.34 U$76.35 U$76.36 U$76.P$1 U$76.P$2 U$76.P$3 U$76.P$4 U$76.P$5 U$76.P$6 U$76.P$7 U$76.P$8 U$76.P$9 U$76.P$10 U$76.P$11 U$76.P$12 U$76.P$13 U$76.P$14 U$76.P$15 U$76.P$16 U$76.P$17 U$76.P$18 U$76.P$19 U$76.P$20 U$76.P$21 U$76.P$22 U$76.P$23 U$76.P$24 U$76.P$25 U$76.P$26 U$76.P$27 U$76.P$28 U$76.P$29 U$76.P$30 U$76.P$31 U$76.P$32 U$77.33 U$77.34 U$77.35 U$77.36 U$77.P$1 U$77.P$2 U$77.P$3 U$77.P$4 U$77.P$5 U$77.P$6 U$77.P$7 U$77.P$8 U$77.P$9 U$77.P$10 U$77.P$11 U$77.P$12 U$77.P$13 U$77.P$14 U$77.P$15 U$77.P$16 U$77.P$17 U$77.P$18 U$77.P$19 U$77.P$20 U$77.P$21 U$77.P$22 U$77.P$23 U$77.P$24 U$77.P$25 U$77.P$26 U$77.P$27 U$77.P$28 U$77.P$29 U$77.P$30 U$77.P$31 U$77.P$32 U$78.33 U$78.34 U$78.35 U$78.36 U$78.P$1 U$78.P$2 U$78.P$3 U$78.P$4 U$78.P$5 U$78.P$6 U$78.P$7 U$78.P$8 U$78.P$9 U$78.P$10 U$78.P$11 U$78.P$12 U$78.P$13 U$78.P$14 U$78.P$15 U$78.P$16 U$78.P$17 U$78.P$18 U$78.P$19 U$78.P$20 U$78.P$21 U$78.P$22 U$78.P$23 U$78.P$24 U$78.P$25 U$78.P$26 U$78.P$27 U$78.P$28 U$78.P$29 U$78.P$30 U$78.P$31 U$78.P$32 U$79.33 U$79.34 U$79.35 U$79.36 U$79.P$1 U$79.P$2 U$79.P$3 U$79.P$4 U$79.P$5 U$79.P$6 U$79.P$7 U$79.P$8 U$79.P$9 U$79.P$10 U$79.P$11 U$79.P$12 U$79.P$13 U$79.P$14 U$79.P$15 U$79.P$16 U$79.P$17 U$79.P$18 U$79.P$19 U$79.P$20 U$79.P$21 U$79.P$22 U$79.P$23 U$79.P$24 U$79.P$25 U$79.P$26 U$79.P$27 U$79.P$28 U$79.P$29 U$79.P$30 U$79.P$31 U$79.P$32 U$80.33 U$80.34 U$80.35 U$80.36 U$80.P$1 U$80.P$2 U$80.P$3 U$80.P$4 U$80.P$5 U$80.P$6 U$80.P$7 U$80.P$8 U$80.P$9 U$80.P$10 U$80.P$11 U$80.P$12 U$80.P$13 U$80.P$14 U$80.P$15 U$80.P$16 U$80.P$17 U$80.P$18 U$80.P$19 U$80.P$20 U$80.P$21 U$80.P$22 U$80.P$23 U$80.P$24 U$80.P$25 U$80.P$26 U$80.P$27 U$80.P$28 U$80.P$29 U$80.P$30 U$80.P$31 U$80.P$32 U$81.33 U$81.34 U$81.35 U$81.36 U$81.P$1 U$81.P$2 U$81.P$3 U$81.P$4 U$81.P$5 U$81.P$6 U$81.P$7 U$81.P$8 U$81.P$9 U$81.P$10 U$81.P$11 U$81.P$12 U$81.P$13 U$81.P$14 U$81.P$15 U$81.P$16 U$81.P$17 U$81.P$18 U$81.P$19 U$81.P$20 U$81.P$21 U$81.P$22 U$81.P$23 U$81.P$24 U$81.P$25 U$81.P$26 U$81.P$27 U$81.P$28 U$81.P$29 U$81.P$30 U$81.P$31 U$81.P$32 U$82.33 U$82.34 U$82.35 U$82.36 U$82.P$1 U$82.P$2 U$82.P$3 U$82.P$4 U$82.P$5 U$82.P$6 U$82.P$7 U$82.P$8 U$82.P$9 U$82.P$10 U$82.P$11 U$82.P$12 U$82.P$13 U$82.P$14 U$82.P$15 U$82.P$16 U$82.P$17 U$82.P$18 U$82.P$19 U$82.P$20 U$82.P$21 U$82.P$22 U$82.P$23 U$82.P$24 U$82.P$25 U$82.P$26 U$82.P$27 U$82.P$28 U$82.P$29 U$82.P$30 U$82.P$31 U$82.P$32 U$83.33 U$83.34 U$83.35 U$83.36 U$83.P$11 U$83.P$22 U$83.P$23 U$83.P$24 U$83.P$25 U$83.P$26 U$83.P$27 U$83.P$28 U$83.P$29 U$83.P$30 U$83.P$31 U$83.P$32 U$84.33 U$84.34 U$84.35 U$84.36 U$84.P$11 U$84.P$22 U$84.P$23 U$84.P$24 U$84.P$25 U$84.P$26 U$84.P$27 U$84.P$28 U$84.P$29 U$84.P$30 U$84.P$31 U$84.P$32

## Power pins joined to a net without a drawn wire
3,3V: USBMODUL.+3,3V(3,3V)

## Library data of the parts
AGND ANT = pinhead:PINHD-1X1: PIN HEADER
C1 C2 = rcl:CPOL-EU: POLARIZED CAPACITOR, European symbol
C3-C8 = rcl:C-EU: CAPACITOR, European symbol
FUNK = RoboterNetzNeu:RFM12: Funkmodul RFM12 (siehe roboternetz.de / robotikhardware.de)
IC1 = RoboterNetzNeu:MEGA32BAUFORM
IC2 = RoboterNetzNeu:LD1117
ISP = RoboterNetzNeu:ISPSTECKER
J1-J4 = RoboterNetzNeu:AST021-10
L1 = rcl:L-EU: INDUCTOR, European symbol
LED1 = led:LED: LED
POW = pinhead:PINHD-1X2: PIN HEADER
POWER = jumper:JP2E: JUMPER
Q1 = crystal:CRYTAL: CRYSTAL
R1-R3 = rcl:R-EU_: RESISTOR, European symbol
U$1-U$24 = RoboterNetzNeu:LOCHRASTER38PIN
U$25-U$42 = RoboterNetzNeu:LOCHRASTER5PIN
U$67-U$84 = RoboterNetzNeu:LOCHRASTER37PIN
USBMODUL = RoboterNetzNeu:USBMODUL_RN_BUCHSE: Buchse oder Stiftleiste zum Anschluss des USBMODULS (Bezug Robotikhardware.de)

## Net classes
0 default: width 0.305 mm
1 Power: width 0.406 mm
2 SuperPower: width 0.61 mm
3 Dick: width 0.813 mm

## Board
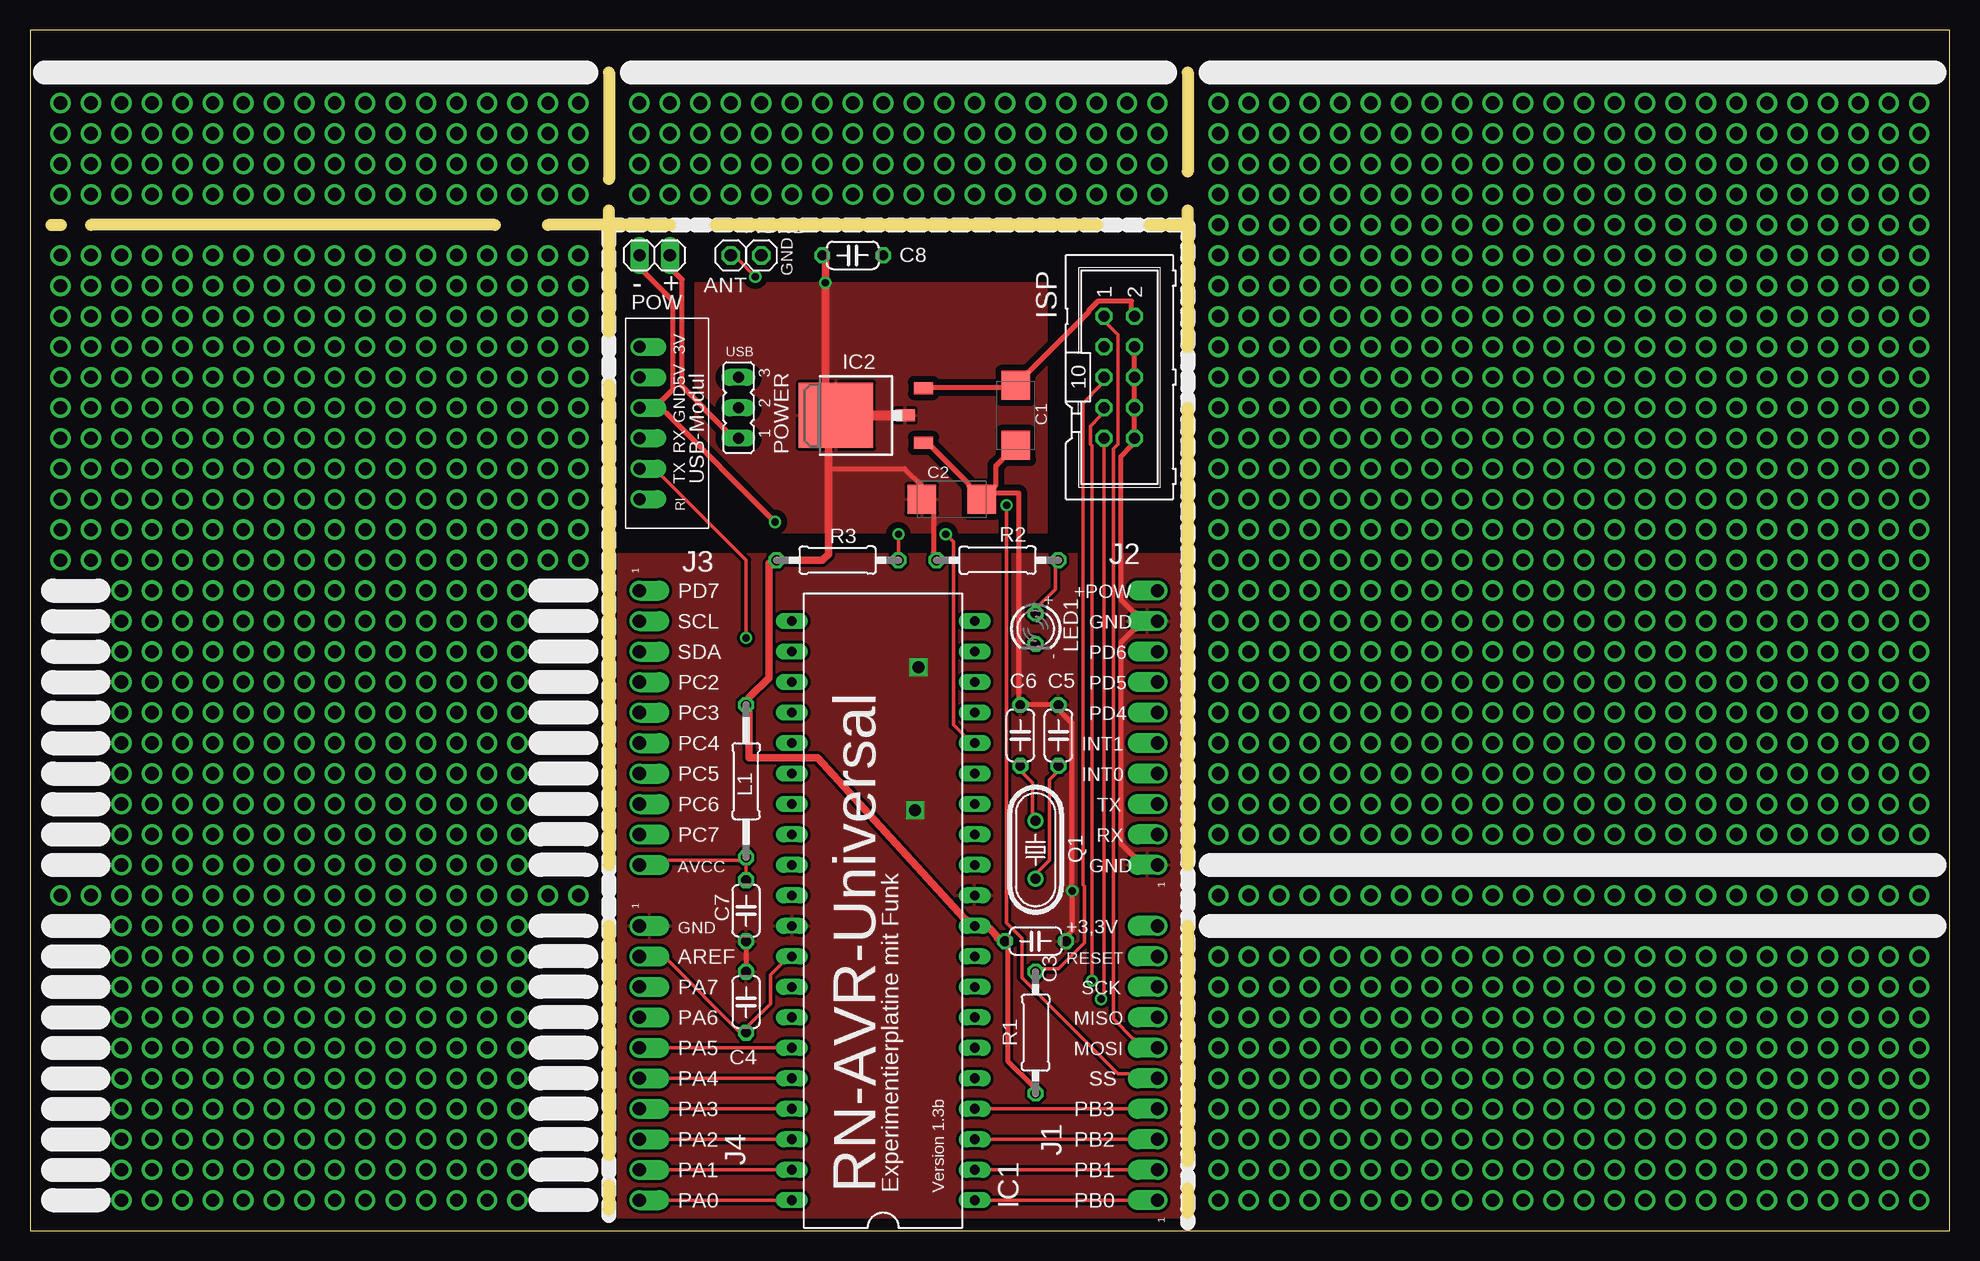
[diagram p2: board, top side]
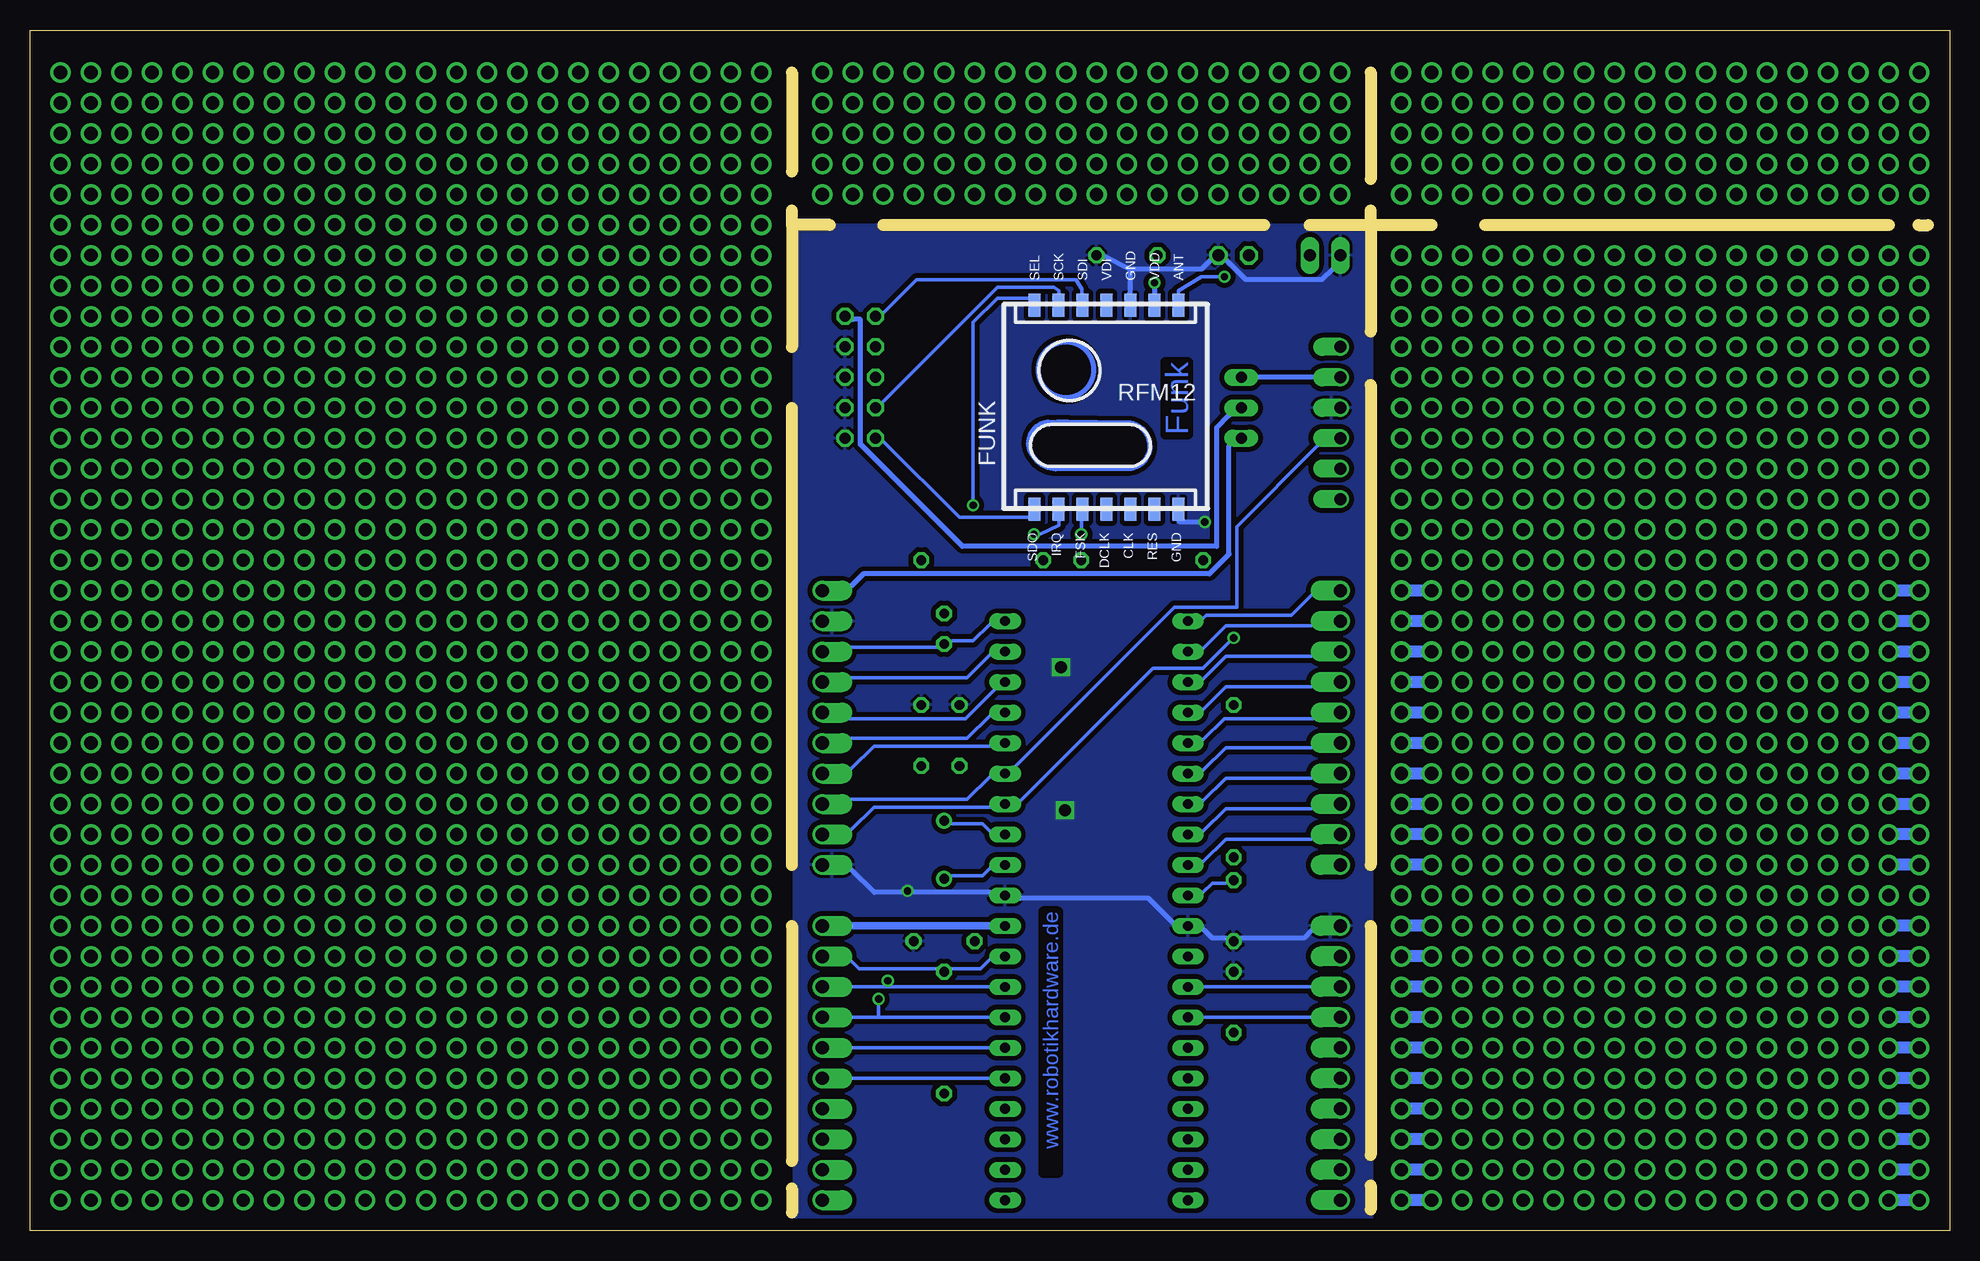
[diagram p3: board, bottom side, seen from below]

Size 160.02 x 100.06 mm. Coordinates in mm from the lower left corner, seen from the top.
Outline: 0,0 160,0 160.02,100.06 0,100.06 0,0
Copper layers (1*16): Top 0.035mm / dielectric 1.5mm / Bottom 0.035mm
Design rules "default *": minimum track width 10mil, minimum drill 24mil, track to track 10mil, track to pad 11mil, pad to pad 11mil, via to via 8mil, smd to smd 12mil, copper to edge 40mil, drill to drill 8mil, minimum pad ring 10mil, minimum via ring 8mil, stop-mask expansion 4mil, vias tented up to drill 0mil, thermal gap 10mil
Milling: 18 lines

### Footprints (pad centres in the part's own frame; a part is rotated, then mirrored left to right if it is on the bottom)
1X01 = drill 1.016 octagon: 1 0,0
SMC_C = smd 2.4 x 2.4: + -2.5,0; - 2.5,0
C050-024X044 = drill 0.813 octagon: 1 -2.54,0; 2 2.54,0
RFM12_SMD = smd 0.965 x 1.93: +3,3V 0,5.5; ANT 2,5.5; CLK -2,-11.5; DCLK -4,-11.5; FSK -6,-11.5; GND@1 2,-11.5; GND@2 -2,5.5; IRQ -8,-11.5; RES 0,-11.5; SCK -8,5.5; SDI -6,5.5; SDO -10,-11.5; SEL -10,5.5; VDI -4,5.5
DIL40 = drill 0.813 long: 1 -22.86,-7.62; 2 -20.32,-7.62; 3 -17.78,-7.62; 4 -15.24,-7.62; 5 -12.7,-7.62; 6 -10.16,-7.62; 7 -7.62,-7.62; 8 -5.08,-7.62; 9 -2.54,-7.62; 10 0,-7.62; 11 2.54,-7.62; 12 5.08,-7.62; 13 7.62,-7.62; 14 10.16,-7.62; 15 12.7,-7.62; 16 15.24,-7.62; 17 17.78,-7.62; 18 20.32,-7.62; 19 22.86,-7.62; 20 25.4,-7.62; 21 25.4,7.62; 22 22.86,7.62; 23 20.32,7.62; 24 17.78,7.62; 25 15.24,7.62; 26 12.7,7.62; 27 10.16,7.62; 28 7.62,7.62; 29 5.08,7.62; 30 2.54,7.62; 31 0,7.62; 32 -2.54,7.62; 33 -5.08,7.62; 34 -7.62,7.62; 35 -10.16,7.62; 36 -12.7,7.62; 37 -15.24,7.62; 38 -17.78,7.62; 39 -20.32,7.62; 40 -22.86,7.62
TO252 = smd 1 x 1.6: 1 -2.28,-4.8; 2 -0.006,-3.276; 3 2.28,-4.8 | smd 5.4 x 6.2: 4 0,2.5
ML10 = drill 0.914 octagon: 1 -5.08,-1.27; 2 -5.08,1.27; 3 -2.54,-1.27; 4 -2.54,1.27; 5 0,-1.27; 6 0,1.27; 7 2.54,-1.27; 8 2.54,1.27; 9 5.08,-1.27; 10 5.08,1.27
AST021-10PIN = drill 1.1 offset: 1 -11.43,0; 2 -8.89,0; 3 -6.35,0; 4 -3.81,0; 5 -1.27,0; 6 1.27,0; 7 3.81,0; 8 6.35,0; 9 8.89,0; 10 11.43,0
0207/12 = drill 0.813 octagon: 1 -6.35,0; 2 6.35,0
LED3MM = drill 0.813 octagon: A -1.27,0; K 1.27,0
1X02 = drill 1.016 long: 1 -1.27,0; 2 1.27,0
JP2 = drill 0.914 long: 1 -2.54,0; 2 0,0; 3 2.54,0
HC49/S = drill 0.813: 1 -2.413,0; 2 2.413,0
0207/10 = drill 0.813 octagon: 1 -5.08,0; 2 5.08,0
LOCHRASTER38PIN = drill 1.1 pad 1.7: P$1 -40.64,0; P$2 -38.1,0; P$3 -35.56,0; P$4 -33.02,0; P$5 -30.48,0; P$6 -27.94,0; P$7 -25.4,0; P$8 -22.86,0; P$9 -20.32,0; P$10 -17.78,0; P$11 -15.24,0; P$12 -12.7,0; P$13 -10.16,0; P$14 -7.62,0; P$15 -5.08,0; P$16 -2.54,0; P$17 0,0; P$18 2.54,0; P$19 5.08,0; P$20 7.62,0; P$21 10.16,0; P$22 12.7,0; P$23 15.24,0; P$24 17.78,0; P$25 20.32,0; P$26 22.86,0; P$27 25.4,0; P$28 27.94,0; P$29 30.48,0; P$30 33.02,0; P$31 35.56,0; P$32 38.1,0; P$33 40.64,0; P$34 43.18,0; P$35 45.72,0; P$36 48.26,0; P$37 50.8,0; P$38 53.34,0
LOACHRASTER5PIN = drill 1.1 pad 1.7: 1 -5.08,0; 2 -2.54,0; 3 0,0; 4 2.54,0; 5 5.08,0
LOCHRASTER37PIN = drill 1.1 pad 1.7: 33 83.82,0; 34 86.36,0; 35 88.9,0; 36 91.44,0; 37 93.98,0; P$1 0,0; P$2 2.54,0; P$3 5.08,0; P$4 7.62,0; P$5 10.16,0; P$6 12.7,0; P$7 15.24,0; P$8 17.78,0; P$9 20.32,0; P$10 22.86,0; P$11 25.4,0; P$12 27.94,0; P$13 30.48,0; P$14 33.02,0; P$15 35.56,0; P$16 38.1,0; P$17 40.64,0; P$18 43.18,0; P$19 45.72,0; P$20 48.26,0; P$21 50.8,0; P$22 53.34,0; P$23 55.88,0; P$24 58.42,0; P$25 60.96,0; P$26 63.5,0; P$27 66.04,0; P$28 68.58,0; P$29 71.12,0; P$30 73.66,0; P$31 76.2,0; P$32 78.74,0
USBMODUL_RN_STECKER = drill 1 offset: +3,3V -6.35,-1.27; +VBUS -3.81,-1.27; GND2 -1.27,-1.27; RI 6.35,-1.27; RXD 1.27,-1.27; TXD 3.81,-1.27

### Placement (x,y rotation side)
AGND  60.96,81.28 0 top
ANT  58.42,81.28 180 top
C1  82.17,67.94 270 top
C2  76.83,60.96 0 top
C3  83.82,24.13 180 top
C4  59.69,19.05 90 top
C5  85.72,41.27 270 top
C6  82.55,41.27 270 top
C7  59.69,26.67 90 top
C8  68.58,81.28 180 top
FUNK  66.29,71.63 0 bottom
IC1  71.12,25.4 90 top
IC2  69.68,67.94 90 top
ISP  90.81,71.12 270 top
J1  93.98,13.97 90 top
J2  93.98,41.91 90 top
J3  50.8,41.91 270 top
J4  50.8,13.97 270 top
L1  59.69,37.47 270 top
LED1  83.82,50.16 270 top
POW  52.07,81.28 180 top
POWER  59.05,68.58 90 top
Q1  83.82,31.75 270 top
R1  83.82,16.51 90 top
R2  80.64,55.88 0 top
R3  67.31,55.88 180 top
U$1  99.06,43.18 90 top
U$2  101.6,43.18 90 top
U$3  104.14,43.18 90 top
U$4  106.68,43.18 90 top
U$5  109.22,43.18 90 top
U$6  111.76,43.18 90 top
U$7  114.3,43.18 90 top
U$8  116.84,43.18 90 top
U$9  119.38,43.18 90 top
U$10  121.92,43.18 90 top
U$11  124.46,43.18 90 top
U$12  127,43.18 90 top
U$13  129.54,43.18 90 top
U$14  132.08,43.18 90 top
U$15  134.62,43.18 90 top
U$16  137.16,43.18 90 top
U$17  139.7,43.18 90 top
U$18  142.24,43.18 90 top
U$19  144.78,43.18 90 top
U$20  147.32,43.18 90 top
U$21  149.86,43.18 90 top
U$22  152.4,43.18 90 top
U$23  154.94,43.18 90 top
U$24  157.48,43.18 90 top
U$25  50.8,91.44 90 top
U$26  53.34,91.44 90 top
U$27  55.88,91.44 90 top
U$28  58.42,91.44 90 top
U$29  60.96,91.44 90 top
U$30  63.5,91.44 90 top
U$31  66.04,91.44 90 top
U$32  68.58,91.44 90 top
U$33  71.12,91.44 90 top
U$34  73.66,91.44 90 top
U$35  76.2,91.44 90 top
U$36  78.74,91.44 90 top
U$37  81.28,91.44 90 top
U$38  83.82,91.44 90 top
U$39  86.36,91.44 90 top
U$40  88.9,91.44 90 top
U$41  91.44,91.44 90 top
U$42  93.98,91.44 90 top
U$67  2.54,2.54 90 top
U$68  5.08,2.54 90 top
U$69  7.62,2.54 90 top
U$70  10.16,2.54 90 top
U$71  12.7,2.54 90 top
U$72  15.24,2.54 90 top
U$73  17.78,2.54 90 top
U$74  20.32,2.54 90 top
U$75  22.86,2.54 90 top
U$76  25.4,2.54 90 top
U$77  27.94,2.54 90 top
U$78  30.48,2.54 90 top
U$79  33.02,2.54 90 top
U$80  35.56,2.54 90 top
U$81  38.1,2.54 90 top
U$82  40.64,2.54 90 top
U$83  43.18,2.54 90 top
U$84  45.72,2.54 90 top
USBMODUL  52.07,67.31 270 top

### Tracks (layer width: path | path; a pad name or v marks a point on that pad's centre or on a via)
+3V3  (via drill 0.61)
  Top 0.406: IC2.4 66.29,67.94 66.29,67.82 66.55,67.56 | 66.55,63.5 72.9,63.5 74.33,62.06 C2.+ 75.31,59.82 75.31,56.52 R2.1 | 80.64,24.38 80.64,24.51 | R1.1 83.57,12.06 81.53,14.1 81.53,23.5 C3.2 | 59.94,43.18 L1.1
  Top 0.61: 66.29,67.94 v66.29,78.99 66.29,81.03 C8.2 | 66.55,67.56 66.55,63.5 66.55,56.39 66.04,55.88 R3.2 61.59,55.63 61.59,46.1 59.94,44.45 L1.1 | 80.64,24.51 80.01,25.15 IC1.10 77.85,26.04 65.66,39.4 59.94,39.4 59.94,43.18 | C3.2 80.64,24.38
  Top 0.813: IC2.2 IC2.4
  Bottom 0.406: v66.29,78.99 FUNK.+3,3V
  Bottom 0.61: IC1.10 J1.10
  pour Top (isolate 0.508): 55.47,78.94 84.73,78.94 84.73,58.22 55.47,58.22
+UB
  Top 0.406: IC2.3 75.18,70.23 81.03,70.23 C1.+ 83.31,71.63 88.27,76.58 88.27,76.71 89.03,77.47 91.82,77.47 91.82,76.83 ISP.2
  Bottom 0.406: POWER.2 60.07,67.94 61.09,66.93 61.09,57.02 82.3,57.02 90.81,65.53 90.81,75.95 91.44,75.95 ISP.2
AREF
  Top 0.305: IC1.32 62.61,22.23 61.72,21.34 61.72,18.92 59.94,17.14 C4.1 59.05,16.64 53.21,22.48 J4.2
AVCC
  Top 0.305: C7.2 L1.2 59.05,30.86 53.21,30.86 J3.10
  Bottom 0.305: IC1.30 62.23,28.19 61.47,28.96 60.33,28.96 C7.2
GND  (via drill 0.61, 1)
  Top 0.406: v62.1,59.05 52.96,68.2 USBMODUL.GND2 52.7,69.22 53.59,70.1 53.59,77.47 51.18,79.88 POW.2 | IC2.1 75.18,65.28 78.23,62.23 78.23,62.1 C2.- | C1.- 81.03,64.26 80.52,63.75 80.52,62.1 C2.- | C3.1 86.61,24.77 86.87,25.02 v86.87,28.32 86.87,42.29 85.98,43.18 C5.1 C6.1 82.42,44.45 82.42,61.47 80.52,61.47 C2.- | ISP.4 ISP.6 ISP.8 ISP.10 91.82,65.41 90.93,64.52 90.93,52.58 91.95,51.56 J2.9 91.95,50.04 90.93,49.02 90.93,32.26 91.95,31.24 J2.1 | C7.1 C4.2
  Bottom 0.406: v62.1,59.05 64.16,59.05 64.29,59.18 FUNK.GND@1 | 68.35,80.11 70.46,81.2 C8.1 | 68.35,80.11 68.35,78.13 FUNK.GND@2 | POW.2 51.44,80.14 52.32,79.25 58.67,79.25 60.33,80.9 AGND.1 61.59,80.9 62.36,80.14 67.56,80.14 68.35,80.11 | J4.1 53.21,25.02 53.85,24.38 59.05,24.38 C7.1 60.33,24.38 61.47,24.38 62.23,25.15 IC1.31 64.77,25.65 66.8,27.69 77.47,27.69 IC1.11 80.01,28.19 86.87,28.19 | 86.87,28.19 89.66,28.19 91.57,30.1 J2.1 | 86.87,28.19 v86.87,28.32
  other vias: 73.76,35.05 74.07,46.94
  pour Top: 49.07,56.39 96.32,56.39 96.32,0.61 49.07,0.61
  pour Bottom (isolate 0.406): 48.16,83.82 96.32,83.82 96.32,0.91 48.16,0.91
INT0  (via drill 0.61)
  Top 0.305: v76.33,58.04 76.96,57.4 76.96,42.16 77.85,41.27 IC1.16
  Bottom 0.305: v76.33,58.04 75.82,58.04 74.27,58.78 FUNK.IRQ | J2.4 91.57,38.48 89.66,40.39 80.01,40.39 IC1.16
INT1
  Bottom 0.305: IC1.17 80.01,42.93 81.92,41.02 91.57,41.02 J2.5
MISO  (via drill 0.61)
  Top 0.305: v89.28,19.3 89.53,19.56 ISP.9
  Bottom 0.305: IC1.7 89.28,17.78 | 89.28,17.78 J1.7 | FUNK.SDO 76.71,59.44 82.55,59.44 88.9,65.79 ISP.9 | 89.28,17.78 v89.28,19.3
MOSI
  Top 0.305: J1.6 91.95,16 90.3,17.65 90.3,65.15 90.68,65.53 90.68,74.68 89.79,75.56 ISP.1
  Bottom 0.305: IC1.6 J1.6 | FUNK.SDI 72.31,78.44 72.82,79.25 86.11,79.25 88.9,76.45 ISP.1
N$1  (via drill 0.61)
  Top 0.305: v60.45,79.5 59.05,80.9 ANT.1
  Bottom 0.305: v60.45,79.5 62.36,79.5 64.29,78.33 FUNK.ANT
N$2  (via drill 0.61)
  Top 0.305: R3.1 v72.39,58.04
  Bottom 0.305: v72.39,58.04 72.39,59.18 FUNK.FSK
N$3
  Top 0.61: U$24.P$10 U$23.P$10 U$22.P$10 U$21.P$10 U$20.P$10 U$19.P$10 U$18.P$10 U$17.P$10 U$16.P$10 U$15.P$10 U$14.P$10 U$13.P$10 U$12.P$10 U$11.P$10 U$10.P$10 U$9.P$10 U$8.P$10 U$7.P$10 U$6.P$10 U$5.P$10 U$4.P$10 U$3.P$10 U$2.P$10 U$1.P$10
N$4
  Bottom 0.406: USBMODUL.+VBUS POWER.3
N$5  (1 unrouted)
  Bottom 0.406: 74.45,67.36 73.46,67.36 68.58,67.31 arc90 66.67,65.41 arc90 68.58,63.5 74.3,63.5 arc90 76.78,65.66 | 74.62,67.36 75.08,67.36 arc-90 76.76,65.68
N$6
  Top 0.305: LED1.A 84.07,52.07 85.47,53.47 85.47,55.24 R2.2
N$7
  Bottom 1.016: U$83.P$1 U$84.P$1
N$8
  Bottom 1.016: U$83.P$2 U$84.P$2
N$9
  Top 0.61: U$24.P$12 U$23.P$12 U$22.P$12 U$21.P$12 U$20.P$12 U$19.P$12 U$18.P$12 U$17.P$12 U$16.P$12 U$15.P$12 U$14.P$12 U$13.P$12 U$12.P$12 U$11.P$12 U$10.P$12 U$9.P$12 U$8.P$12 U$7.P$12 U$6.P$12 U$5.P$12 U$4.P$12 U$3.P$12 U$2.P$12 U$1.P$12
N$10
  Bottom 1.016: U$83.P$3 U$84.P$3
N$11
  Bottom 1.016: U$83.P$4 U$84.P$4
N$12
  Bottom 1.016: U$83.P$5 U$84.P$5
N$13
  Bottom 1.016: U$83.P$6 U$84.P$6
N$14
  Bottom 1.016: U$83.P$7 U$84.P$7
N$15
  Bottom 1.016: U$83.P$8 U$84.P$8
N$16
  Bottom 1.016: U$83.P$9 U$84.P$9
N$17
  Bottom 1.016: U$83.P$10 U$84.P$10
N$18
  Bottom 1.016: U$83.P$12 U$84.P$12
N$19
  Bottom 1.016: U$83.P$13 U$84.P$13
N$20
  Bottom 1.016: U$83.P$14 U$84.P$14
N$21
  Top 0.61: U$84.37 U$83.37 U$82.37 U$81.37 U$80.37 U$79.37 U$78.37 U$77.37 U$76.37 U$75.37 U$74.37 U$73.37 U$72.37 U$71.37 U$70.37 U$69.37 U$68.37 U$67.37
N$22
  Bottom 1.016: U$83.P$15 U$84.P$15
N$23
  Bottom 1.016: U$83.P$16 U$84.P$16
N$24
  Bottom 1.016: U$83.P$17 U$84.P$17
N$25
  Top 0.305: U$42.5 U$41.5 U$40.5 U$39.5 U$38.5 U$37.5 U$36.5 U$35.5 U$34.5 U$33.5 U$32.5 U$31.5 U$30.5 U$29.5 U$28.5 U$27.5 U$26.5 U$25.5
N$26
  Bottom 1.016: U$83.P$18 U$84.P$18
N$27
  Bottom 1.016: U$83.P$19 U$84.P$19
N$28
  Top 0.61: U$24.P$38 U$23.P$38 U$22.P$38 U$21.P$38 U$20.P$38 U$19.P$38 U$18.P$38 U$17.P$38 U$16.P$38 U$15.P$38 U$14.P$38 U$13.P$38 U$12.P$38 U$11.P$38 U$10.P$38 U$9.P$38 U$8.P$38 U$7.P$38 U$6.P$38 U$5.P$38 U$4.P$38 U$3.P$38 U$2.P$38 U$1.P$38
N$29
  Bottom 1.016: U$83.P$20 U$84.P$20
N$30
  Bottom 1.016: U$83.P$21 U$84.P$21
N$31
  Bottom 1.016: U$67.P$1 U$68.P$1
N$32
  Bottom 1.016: U$67.P$2 U$68.P$2
N$33
  Bottom 1.016: U$67.P$3 U$68.P$3
N$34
  Bottom 1.016: U$67.P$4 U$68.P$4
N$35
  Bottom 1.016: U$67.P$5 U$68.P$5
N$36
  Bottom 1.016: U$67.P$6 U$68.P$6
N$37
  Bottom 1.016: U$67.P$7 U$68.P$7
N$38
  Bottom 1.016: U$67.P$8 U$68.P$8
N$39
  Bottom 1.016: U$67.P$9 U$68.P$9
N$40
  Bottom 1.016: U$67.P$10 U$68.P$10
N$41
  Bottom 1.016: U$67.P$12 U$68.P$12
N$42
  Bottom 1.016: U$67.P$13 U$68.P$13
N$43
  Bottom 1.016: U$67.P$14 U$68.P$14
N$44
  Bottom 1.016: U$67.P$15 U$68.P$15
N$45
  Bottom 1.016: U$67.P$16 U$68.P$16
N$46
  Bottom 1.016: U$67.P$17 U$68.P$17
N$47
  Bottom 1.016: U$67.P$18 U$68.P$18
N$48
  Bottom 1.016: U$67.P$19 U$68.P$19
N$49
  Bottom 1.016: U$67.P$20 U$68.P$20
N$50
  Bottom 1.016: U$67.P$21 U$68.P$21
PA0
  Top 0.305: J4.10 IC1.40
PA1
  Top 0.305: J4.9 IC1.39
PA2
  Top 0.305: J4.8 IC1.38
PA3
  Top 0.305: J4.7 IC1.37
PA4
  Top 0.305: J4.6 IC1.36
PA5
  Top 0.305: J4.5 IC1.35
PA6
  Bottom 0.305: J4.4 IC1.34
PA7
  Bottom 0.305: J4.3 IC1.33
PB0
  Top 0.305: IC1.1 J1.1
PB1
  Top 0.305: IC1.2 J1.2
PB2
  Top 0.305: IC1.3 J1.3
PB3
  Top 0.305: IC1.4 J1.4
PC2
  Bottom 0.305: IC1.24 62.23,43.43 60.33,45.34 53.21,45.34 J3.4
PC3
  Bottom 0.305: IC1.25 62.23,40.89 60.45,42.67 53.09,42.67 J3.5
PC4
  Bottom 0.305: IC1.26 62.23,38.35 60.33,40.26 53.21,40.26 J3.6
PC5
  Bottom 0.305: IC1.27 62.23,35.81 60.33,37.72 53.21,37.72 J3.7
PC6
  Bottom 0.305: IC1.28 62.23,33.27 60.33,35.18 53.21,35.18 J3.8
PC7
  Bottom 0.305: IC1.29 62.23,30.73 60.33,32.64 53.21,32.64 J3.9
PD4
  Bottom 0.305: IC1.18 79.63,45.09 82.04,42.67 91.69,42.67 J2.6
PD5
  Bottom 0.305: IC1.19 80.01,48.01 81.92,46.1 91.57,46.1 J2.7
PD6
  Bottom 0.305: IC1.20 80.01,50.55 81.41,49.15 83.19,49.15 LED1.K 84.45,48.64 91.57,48.64 J2.8
PD7
  Bottom 0.305: IC1.21 62.23,51.05 61.98,51.31 54.86,51.31 53.21,52.96 J3.1
RESET
  Top 0.305: ISP.5 89.28,70.48 87.76,68.96 87.76,28.83 87.88,28.7 87.88,24 85.72,21.84 84.45,21.84 R1.2
  Bottom 0.305: IC1.9 80.01,22.61 80.77,21.84 83.19,21.84 R1.2 84.45,21.84 90.93,21.84 91.57,22.48 J1.9
RX  (via drill 0.61)
  Top 0.305: v59.69,49.4 59.69,55.88 52.7,62.87 USBMODUL.TXD
  Bottom 0.305: J2.2 91.57,33.4 89.66,35.31 80.01,35.31 IC1.14 77.47,35.81 66.42,46.86 62.23,46.86 v59.69,49.4
SCK  (via drill 0.61)
  Top 0.305: v88.52,20.83 88.52,65.41 88.39,65.53 88.39,67.06 89.28,67.94 ISP.7
  Bottom 0.305: IC1.8 88.52,20.32 | 88.52,20.32 J1.8 | FUNK.SCK 74.27,78.33 74.65,78.61 79.38,78.61 89.03,68.96 ISP.7 | 88.52,20.32 v88.52,20.83
SCL
  Bottom 0.305: IC1.22 62.23,48.51 60.33,50.42 53.21,50.42 J3.2
SDA
  Bottom 0.305: IC1.23 62.23,45.97 60.33,47.88 53.21,47.88 J3.3
SS  (via drill 0.61)
  Top 0.305: v81.41,60.45 81.41,25.65 82.68,24.38 82.68,21.08 90.68,13.08 91.57,13.08 J1.5
  Bottom 0.305: v81.41,60.45 81.41,75.69 79.38,77.72 76.71,77.72 FUNK.SEL | IC1.5 J1.5
TX
  Bottom 0.305: J2.3 91.57,35.94 81.92,35.94 80.01,37.85 IC1.15 77.85,38.73 64.64,51.94 59.44,51.94 59.44,58.67 52.7,65.41 USBMODUL.RXD
UEINGANG
  Top 0.406: POWER.1 58.04,66.67 54.36,70.36 54.36,79.25 53.72,79.88 POW.1
  Bottom 0.406: J2.10 91.57,53.72 90.55,54.74 61.72,54.74 60.07,56.39 60.07,65.41 POWER.1
XTAL1
  Top 0.305: C6.2 82.8,38.1 83.57,37.34 83.57,34.8 Q1.1
  Bottom 0.305: IC1.13 80.01,33.27 80.64,33.91 83.19,33.91 Q1.1
XTAL2
  Top 0.305: C5.2 85.47,38.1 84.96,37.59 84.96,30.86 84.07,29.97 Q1.2
  Bottom 0.305: IC1.12 80.01,30.23 80.64,29.59 83.19,29.59 Q1.2
(copper drawn outside any net)
  shapes: Bottom circle x1

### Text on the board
Bottom: Funk | www.robotikhardware.de
tPlace: GND | - | + | USB | PD7 | +POW | + | SCL | GND | SDA | - | PD6 | PC2 | PD5 | PC3 | PD4 | PC4 | INT1 | PC5 | INT0 | PC6 | TX | PC7 | RX | AVCC | GND | GND | +3,3V | AREF | RESET | PA7 | SCK | PA6 | MISO | PA5 | MOSI | PA4 | SS | PA3 | PB3 | PA2 | PB2 | PA1 | PB1 | RN-AVR-Universal | Experimentierplatine mit Funk | Version 1.3b | PA0 | PB0
tDocu: Bitte darauf achten das dicke Linien im Layer 21 alle sichtbar sind! Beim letzten mal sind die im Lochrasterbereich nicht erkennbar gewesen!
